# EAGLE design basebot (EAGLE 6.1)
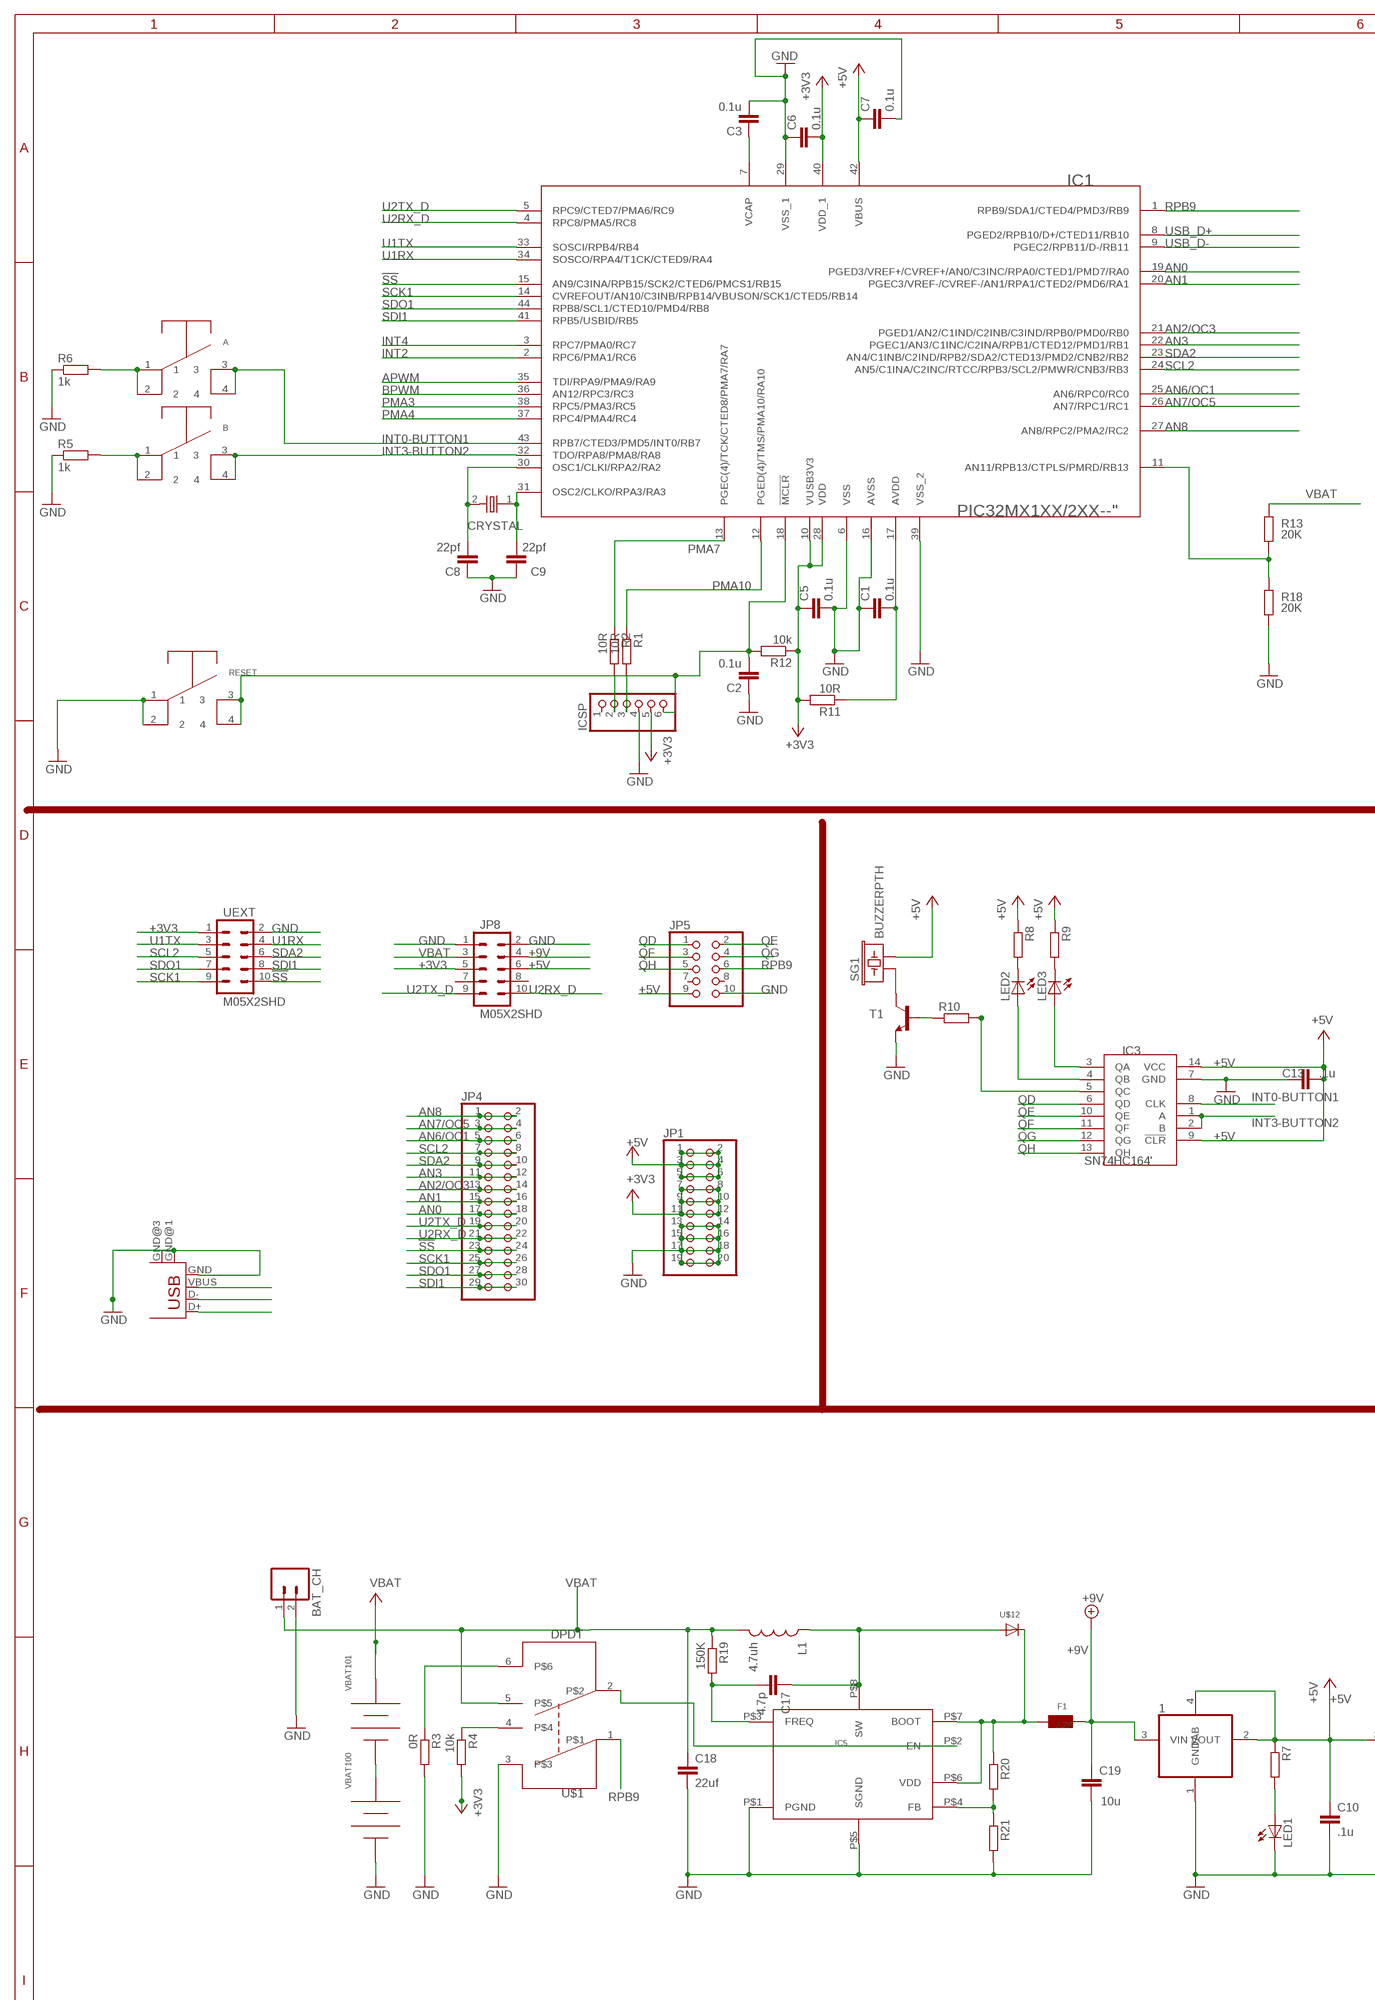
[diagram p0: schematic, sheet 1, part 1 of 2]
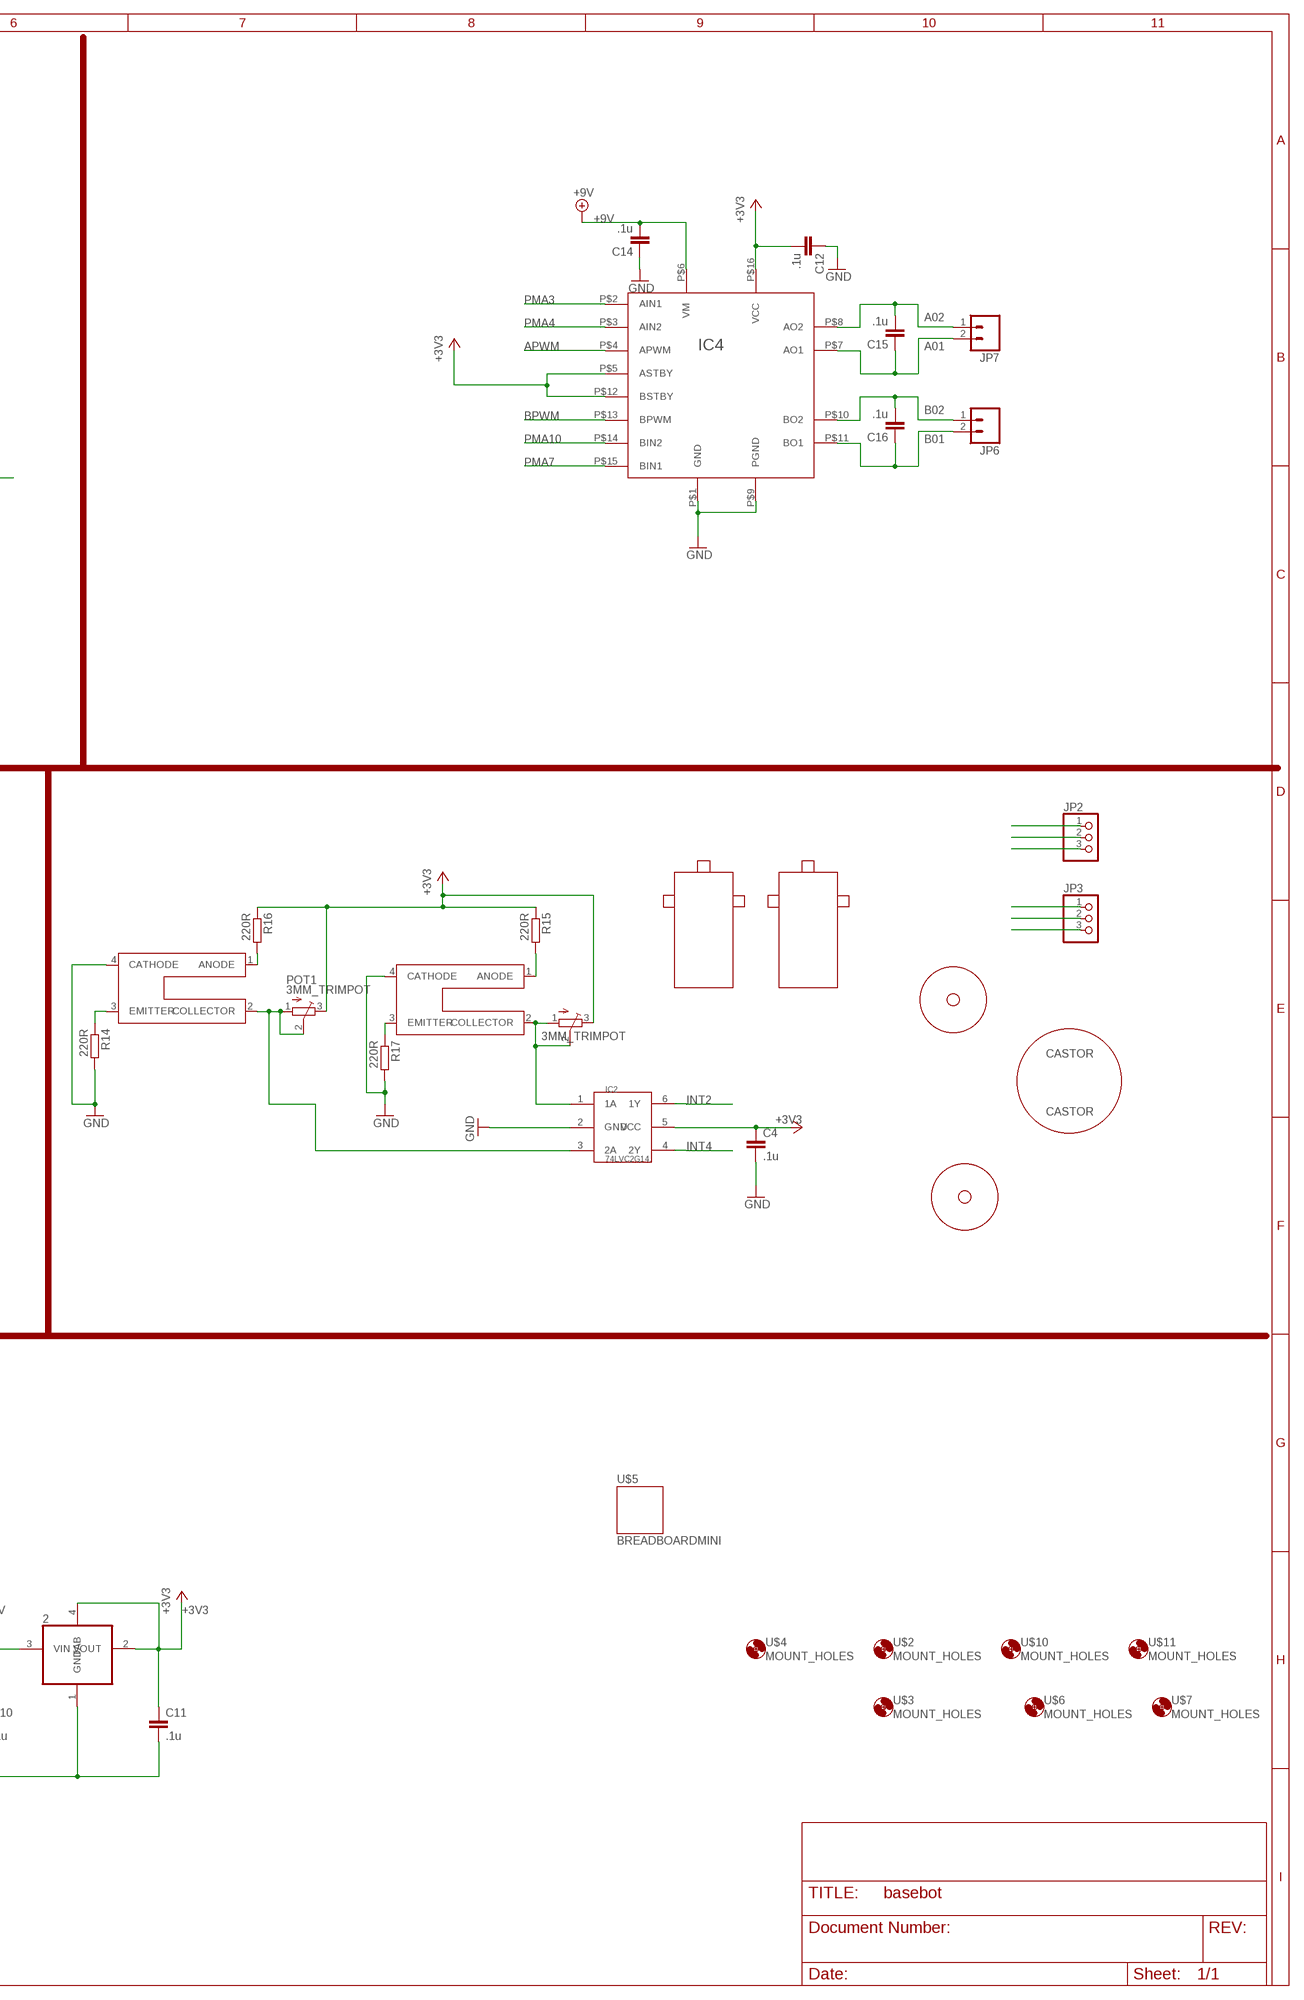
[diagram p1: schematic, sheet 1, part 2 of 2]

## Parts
1  REG1117  [SOT223]
2  REG1117  [SOT223]
A  SWITCH_MOMENTARY  [SWITCH_SMD]
B  SWITCH_MOMENTARY  [SWITCH_SMD]
BAT_CH  M02-JST-2-PTH-NO_SILK  [JST-2-PTH-NS]
C1  0.1u  C-EUC0805  [C0805]
C2  0.1u  C-EUC0805  [C0805]
C3  0.1u  C-EUC0805  [C0805]
C4  .1u  C-EUC0805  [C0805]
C5  0.1u  C-EUC0805  [C0805]
C6  0.1u  C-EUC0805  [C0805]
C7  0.1u  C-EUC0805  [C0805]
C8  22pf  C-EUC0805  [C0805]
C9  22pf  C-EUC0805  [C0805]
C10  .1u  C-EUC0805  [C0805]
C11  .1u  C-EUC0805  [C0805]
C12  .1u  C-EUC0805  [C0805]
C13  .1u  C-EUC0805  [C0805]
C14  .1u  C-EUC0805  [C0805]
C15  .1u  C-EUC0805  [C0805]
C16  .1u  C-EUC0805  [C0805]
C17  4.7p  C-EUC0805  [C0805]
C18  22uf  C-EUC0805  [C0805]
C19  10u  C-EUC0805  [C0805]
CASTOR  CASTOR  [CASTOR-16.66MM]
CRYSTAL  CRYSTAL2PIN  [CRYSTAL-2PIN]
F1  1.2A  PPTC  [PPTC1812]
IC1  PIC32MX1XX/2XX--"  [44TQFP]
IC2  74LVC2G14.  [6TSOP]
IC3  SN74HC164'  [SOIC-14]
IC4  TB6552FN  [16PIN_SSOP]
IC5  LM2623  [MSOP-8L-EDP]
ICSP  PINHD-1X6  [1X06]
JP1  PINHD-2X10  [2X10]
JP2  PINHD-1X3  [1X03]
JP3  PINHD-1X3  [1X03]
JP4  PINHD-2X15  [2X15]
JP5  PINHD-2X5  [2X05]
JP6  M02-JST-2-PTH-NO_SILK  [JST-2-PTH-NS]
JP7  M02-JST-2-PTH-NO_SILK  [JST-2-PTH-NS]
JP8  M05X2SHD  [2X5-SHROUDED]
L1  4.7uh  INDUCTORNPI75  [NPI75C]
LED1  LEDCHIP-LED0805  [CHIP-LED0805]
LED2  LEDCHIP-LED0805  [CHIP-LED0805]
LED3  LEDCHIP-LED0805  [CHIP-LED0805]
LEFT1  DUAL_SHAFT_PLASTIC_GEAR_MOTOR_ST1_LEFT  [DUAL_SHAFT_PLASTIC_GEAR_MOTOR_ST1_LEFT]
POT  3MM_TRIMPOT  [3MM_TRIMPOT]
POT1  3MM_TRIMPOT  [3MM_TRIMPOT]
R1  10R  R-EU_R0805  [R0805]
R2  10R  R-EU_R0805  [R0805]
R3  0R  R-EU_R0805  [R0805]
R4  10k  R-EU_R0805  [R0805]
R5  1k  R-EU_R0805  [R0805]
R6  1k  R-EU_R0805  [R0805]
R7  R-EU_R0805  [R0805]
R8  R-EU_R0805  [R0805]
R9  R-EU_R0805  [R0805]
R10  R-EU_R0805  [R0805]
R11  10R  R-EU_R0805  [R0805]
R12  10k  R-EU_R0805  [R0805]
R13  20K  R-EU_R0805  [R0805]
R14  220R  R-EU_R0805  [R0805]
R15  220R  R-EU_R0805  [R0805]
R16  220R  R-EU_R0805  [R0805]
R17  220R  R-EU_R0805  [R0805]
R18  20K  R-EU_R0805  [R0805]
R19  150K  R-EU_R0805  [R0805]
R20  R-EU_R0805  [R0805]
R21  R-EU_R0805  [R0805]
RESET  SWITCH_MOMENTARY  [SWITCH_SMD]
RIGHT1  DUAL_SHAFT_PLASTIC_GEAR_MOTOR_ST1_RIGHT  [DUAL_SHAFT_PLASTIC_GEAR_MOTOR_ST1_RIGHT]
SG1  BUZZERPTH  [BUZZER-12MM]
T1  MMBT2222ALT1-NPN-SOT23-BEC  [SOT23-BEC]
U$1  DPDT  [DPDT]
U$2  MOUNT_HOLES  [HOLES-1.6MM]
U$3  MOUNT_HOLES  [HOLES-1.6MM]
U$4  MOUNT_HOLES  [HOLES-1.6MM]
U$5  BREADBOARDMINI  [BREADBOARD-MINI]
U$6  MOUNT_HOLES  [HOLES-1.6MM]
U$7  MOUNT_HOLES  [HOLES-1.6MM]
U$8  GP1S092HCPIF  [GP1S092HCPIF]
U$9  GP1S092HCPIF  [GP1S092HCPIF]
U$10  MOUNT_HOLES  [HOLES-1.6MM]
U$11  MOUNT_HOLES  [HOLES-1.6MM]
U$12  DIODESMA  [SMADIODE]
UEXT  M05X2SHD  [2X5-SHROUDED]
USB1  USB-MB-S  [USB-MB-S]
VBAT100  BATTERY_HOLDERAA  [AA_BATTERY_HOLDER]
VBAT101  BATTERY_HOLDERAA  [AA_BATTERY_HOLDER]
WHEEL1  69X8MM-WHEEL  [69X8MM-WHEEL]
WHEEL2  69X8MM-WHEEL  [69X8MM-WHEEL]

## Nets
!SS: IC1.15(AN9/C3INA/RPB15/SCK2/CTED6/PMCS1/RB15) JP4.23 JP4.24 UEXT.10
+3V3: 2.2(VOUT) 2.4(TAB) C4.1 C5.1 C6.2 C11.1 C12.2 IC1.10(VUSB3V3) IC1.28(VDD) IC1.40(VDD_1) IC2.5(VCC) IC4.P$5(ASTBY) IC4.P$12(BSTBY) IC4.P$16(VCC) ICSP.5 JP1.7 JP1.8 JP1.9 JP1.10 JP1.11 JP1.12 JP8.5 POT1.3(E) POT.3(E) R4.2 R11.2 R12.1 R15.1 R16.1 UEXT.1
+5V: 1.2(VOUT) 1.4(TAB) 2.3(VIN) C7.1 C10.1 C13.1 IC1.42(VBUS) IC3.9(!CLR) IC3.14(VCC) JP1.1 JP1.2 JP1.3 JP1.4 JP1.5 JP1.6 JP2.2 JP3.2 JP5.9 JP8.6 R7.1 R8.1 R9.1 SG1.- USB1.VBUS
+9V: 1.3(VIN) C14.2 C19.2 F1.P$2 IC4.P$6(VM) JP8.4
A01: C15.1 IC4.P$7(AO1) JP7.2
A02: C15.2 IC4.P$8(AO2) JP7.1
AN0: IC1.19(PGED3/VREF+/CVREF+/AN0/C3INC/RPA0/CTED1/PMD7/RA0) JP4.17 JP4.18
AN1: IC1.20(PGEC3/VREF-/CVREF-/AN1/RPA1/CTED2/PMD6/RA1) JP4.15 JP4.16
AN2/OC3: IC1.21(PGED1/AN2/C1IND/C2INB/C3IND/RPB0/PMD0/RB0) JP4.13 JP4.14
AN3: IC1.22(PGEC1/AN3/C1INC/C2INA/RPB1/CTED12/PMD1/RB1) JP4.11 JP4.12
AN6/OC1: IC1.25(AN6/RPC0/RC0) JP2.1 JP4.5 JP4.6
AN7/OC5: IC1.26(AN7/RPC1/RC1) JP3.1 JP4.3 JP4.4
AN8: IC1.27(AN8/RPC2/PMA2/RC2) JP4.1 JP4.2
APWM: IC1.35(TDI/RPA9/PMA9/RA9) IC4.P$4(APWM)
B01: C16.1 IC4.P$11(BO1) JP6.2
B02: C16.2 IC4.P$10(BO2) JP6.1
BPWM: IC1.36(AN12/RPC3/RC3) IC4.P$13(BPWM)
GND: 1.1(GND) 2.1(GND) BAT_CH.2 C1.1 C2.1 C3.2 C4.2 C5.2 C6.1 C7.2 C8.1 C9.1 C10.2 C11.2 C12.1 C13.2 C14.1 C18.2 C19.1 IC1.6(VSS) IC1.16(AVSS) IC1.29(VSS_1) IC1.39(VSS_2) IC2.2(GND) IC3.7(GND) IC4.P$1(GND) IC4.P$9(PGND) IC5.P$1(PGND) IC5.P$5(SGND) ICSP.4 JP1.13 JP1.14 JP1.15 JP1.16 JP1.17 JP1.18 JP1.19 JP1.20 JP2.3 JP3.3 JP5.10 JP8.1 JP8.2 LED1.C R3.2 R5.1 R6.1 R14.2 R17.2 R18.2 R21.2 RESET.1 RESET.2 T1.E U$1.3 U$8.4(CATHODE) U$9.4(CATHODE) UEXT.2 USB1.GND USB1.GND@1(GND) USB1.GND@3(GND) VBAT100.-
INT0-BUTTON1: A.3 A.4 IC1.43(RPB7/CTED3/PMD5/INT0/RB7) IC3.8(CLK)
INT2: IC1.2(RPC6/PMA1/RC6) IC2.6(1Y)
INT3-BUTTON2: B.3 B.4 IC1.32(TDO/RPA8/PMA8/RA8) IC3.1(A) IC3.2(B)
INT4: IC1.3(RPC7/PMA0/RC7) IC2.4(2Y)
MCLR: C2.2 IC1.18(!MCLR) ICSP.6 R12.2 RESET.3 RESET.4
N$1: IC1.11(AN11/RPB13/CTPLS/PMRD/RB13) R13.2 R18.1
N$3: C3.1 IC1.7(VCAP)
N$5: C17.2 IC5.P$3(FREQ) R19.2
N$6: LED1.A R7.2
N$7: IC3.3(QA) LED3.A
N$8: IC3.4(QB) LED2.A
N$14: IC3.5(QC) R10.2
N$15: LED3.C R9.2
N$16: LED2.C R8.2
N$17: R10.1 T1.B
N$18: ICSP.3 R1.2
N$19: ICSP.2 R2.2
N$20: VBAT100.+ VBAT101.-
N$22: A.1 A.2 R6.2
N$23: B.1 B.2 R5.2
N$24: R4.1 U$1.4
N$25: R3.1 U$1.6
N$26: SG1.+ T1.C
N$27: C17.1 IC5.P$8(SW) L1.1 U$12.A
N$28: IC5.P$2(EN) U$1.2
N$29: IC5.P$4(FB) R20.2 R21.1
N$30: F1.P$1 IC5.P$6(VDD) IC5.P$7(BOOT) R20.1 U$12.C
N$36: R16.2 U$9.1(ANODE)
N$37: R15.2 U$8.1(ANODE)
N$38: R14.1 U$9.3(EMITTER)
N$39: C8.2 CRYSTAL.2 IC1.30(OSC1/CLKI/RPA2/RA2)
N$40: R17.1 U$8.3(EMITTER)
N$41: C9.2 CRYSTAL.1 IC1.31(OSC2/CLKO/RPA3/RA3)
N$42: IC2.3(2A) POT1.1(A) POT1.2(S) U$9.2(COLLECTOR)
N$44: C1.2 IC1.17(AVDD) R11.1
N$45: IC2.1(1A) POT.1(A) POT.2(S) U$8.2(COLLECTOR)
PMA3: IC1.38(RPC5/PMA3/RC5) IC4.P$2(AIN1)
PMA4: IC1.37(RPC4/PMA4/RC4) IC4.P$3(AIN2)
PMA7: IC1.13(PGEC(4)/TCK/CTED8/PMA7/RA7) IC4.P$15(BIN1) R2.1
PMA10: IC1.12(PGED(4)/TMS/PMA10/RA10) IC4.P$14(BIN2) R1.1
QD: IC3.6(QD) JP5.1
QE: IC3.10(QE) JP5.2
QF: IC3.11(QF) JP5.3
QG: IC3.12(QG) JP5.4
QH: IC3.13(QH) JP5.5
RPB9: IC1.1(RPB9/SDA1/CTED4/PMD3/RB9) JP5.6 U$1.1
SCK1: IC1.14(CVREFOUT/AN10/C3INB/RPB14/VBUSON/SCK1/CTED5/RB14) JP4.25 JP4.26 UEXT.9
SCL2: IC1.24(AN5/C1INA/C2INC/RTCC/RPB3/SCL2/PMWR/CNB3/RB3) JP4.7 JP4.8 UEXT.5
SDA2: IC1.23(AN4/C1INB/C2IND/RPB2/SDA2/CTED13/PMD2/CNB2/RB2) JP4.9 JP4.10 UEXT.6
SDI1: IC1.41(RPB5/USBID/RB5) JP4.29 JP4.30 UEXT.8
SDO1: IC1.44(RPB8/SCL1/CTED10/PMD4/RB8) JP4.27 JP4.28 UEXT.7
U1RX: IC1.34(SOSCO/RPA4/T1CK/CTED9/RA4) UEXT.4
U1TX: IC1.33(SOSCI/RPB4/RB4) UEXT.3
U2RX_D: IC1.4(RPC8/PMA5/RC8) JP4.21 JP4.22 JP8.10
U2TX_D: IC1.5(RPC9/CTED7/PMA6/RC9) JP4.19 JP4.20 JP8.9
USB_D+: IC1.8(PGED2/RPB10/D+/CTED11/RB10) USB1.D+
USB_D-: IC1.9(PGEC2/RPB11/D-/RB11) USB1.D-
VBAT: BAT_CH.1 C18.1 JP8.3 L1.2 R13.1 R19.1 U$1.5 VBAT101.+
Unconnected: ICSP.1 JP5.7 JP5.8 JP8.7 JP8.8

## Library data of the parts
1 2 = BaseApp:REG1117: 800mA and 1A Low Dropout (LDO) Positive Regulator 1.8V, 2.5V, 2.85V, 3.3V, 5V, and Adj http://www.digikey.com/product-detail/en/LM1117MPX-3.3%2FNOPB/LM1117MPX-3.3CT-ND/1010516
A B RESET = BaseApp:SWITCH_MOMENTARY: Soft Switch http://www.digikey.com/product-detail/en/EVQ-Q2B03W/P12932SCT-ND/762922
BAT_CH JP6 JP7 = SparkFun:M02: Header 2
C1-C19 = rcl:C-EU: CAPACITOR, European symbol
CASTOR = BaseApp:CASTOR
CRYSTAL = BaseApp:CRYSTAL: CRYSTAL
F1 = BaseApp:PPTC: PPTC FUSE :- Ih-750ma; It-1.5A; Vmax-40V
IC1 = BaseApp:PIC32MX1XX/2XX--: PIC32MX250F128D-I/PT http://www.digikey.com/product-detail/en/PIC32MX250F128D-I%2FPT/PIC32MX250F128D-I%2FPT-ND/3046589
IC2 = BaseApp:74LVC2G14: 74LVC2G14 :-Dual inverting Schmitt trigger http://www.digikey.com/product-detail/en/74LVC2G14GW,125/568-4840-1-ND/2116536
IC3 = BaseApp:SN74HC164: http://www.digikey.com/product-detail/en/SN74HC164PWR/296-14020-1-ND/522545 http://www.digikey.com/product-detail/en/MC74HC164ADG/MC74HC164ADGOS-ND/1479883
IC4 = BaseApp:TB6552FN
IC5 = BaseApp:LM2623: LM2623 http://www.digikey.com/product-detail/en/LM2623MM%2FNOPB/LM2623MM%2FNOPBCT-ND/483063
ICSP = adafruit:PINHD-1X6: PIN HEADER
JP1 = pinhead:PINHD-2X10: PIN HEADER
JP2 JP3 = adafruit:PINHD-1X3: PIN HEADER
JP4 = pinhead:PINHD-2X15: PIN HEADER
JP5 = pinhead:PINHD-2X5: PIN HEADER
JP8 UEXT = SparkFun:M05X2: Header 5x2 Standard 10-pin dual row 0.1" header. Commonly used with AVR-ISP. Use with Spark Fun Electronics SKU: PRT-00778
L1 = SparkFun:INDUCTOR: Inductors
LED1-LED3 = adafruit:LED: LED
LEFT1 = BaseApp:DUAL_SHAFT_PLASTIC_GEAR_MOTOR_ST1_LEFT
POT POT1 = BaseApp:3MM_TRIMPOT
R1-R21 = rcl:R-EU_: RESISTOR, European symbol
RIGHT1 = BaseApp:DUAL_SHAFT_PLASTIC_GEAR_MOTOR_ST1_RIGHT
SG1 = SparkFun:BUZZER: Buzzer 12mm
T1 = transistor:*-NPN-: NPN Transistror BF959 corrected 2008.03.06
U$1 = BaseApp:DPDT: http://www.digikey.com/product-detail/en/JS202011SCQN/401-2002-1-ND/1640098
U$2-U$4 U$6 U$7 U$10 U$11 = BaseApp:MOUNT_HOLES
U$5 = SparkFun:BREADBOARD: Breadboard Mini Self Adhesive
U$8 U$9 = BaseApp:GP1S092HCPIF: GP1S092HCPIF :- SMT, Gap : 2mm, Slit : 0.3mm Phototransistor Output, Compact Transmissive Photointerrupter
U$12 = BaseApp:DIODE
USB1 = con-usb-2(1):USB: USB Connectors
VBAT100 VBAT101 = BaseApp:BATTERY_HOLDER: BU2032SM-HD-G
WHEEL1 WHEEL2 = BaseApp:69X8MM-WHEEL

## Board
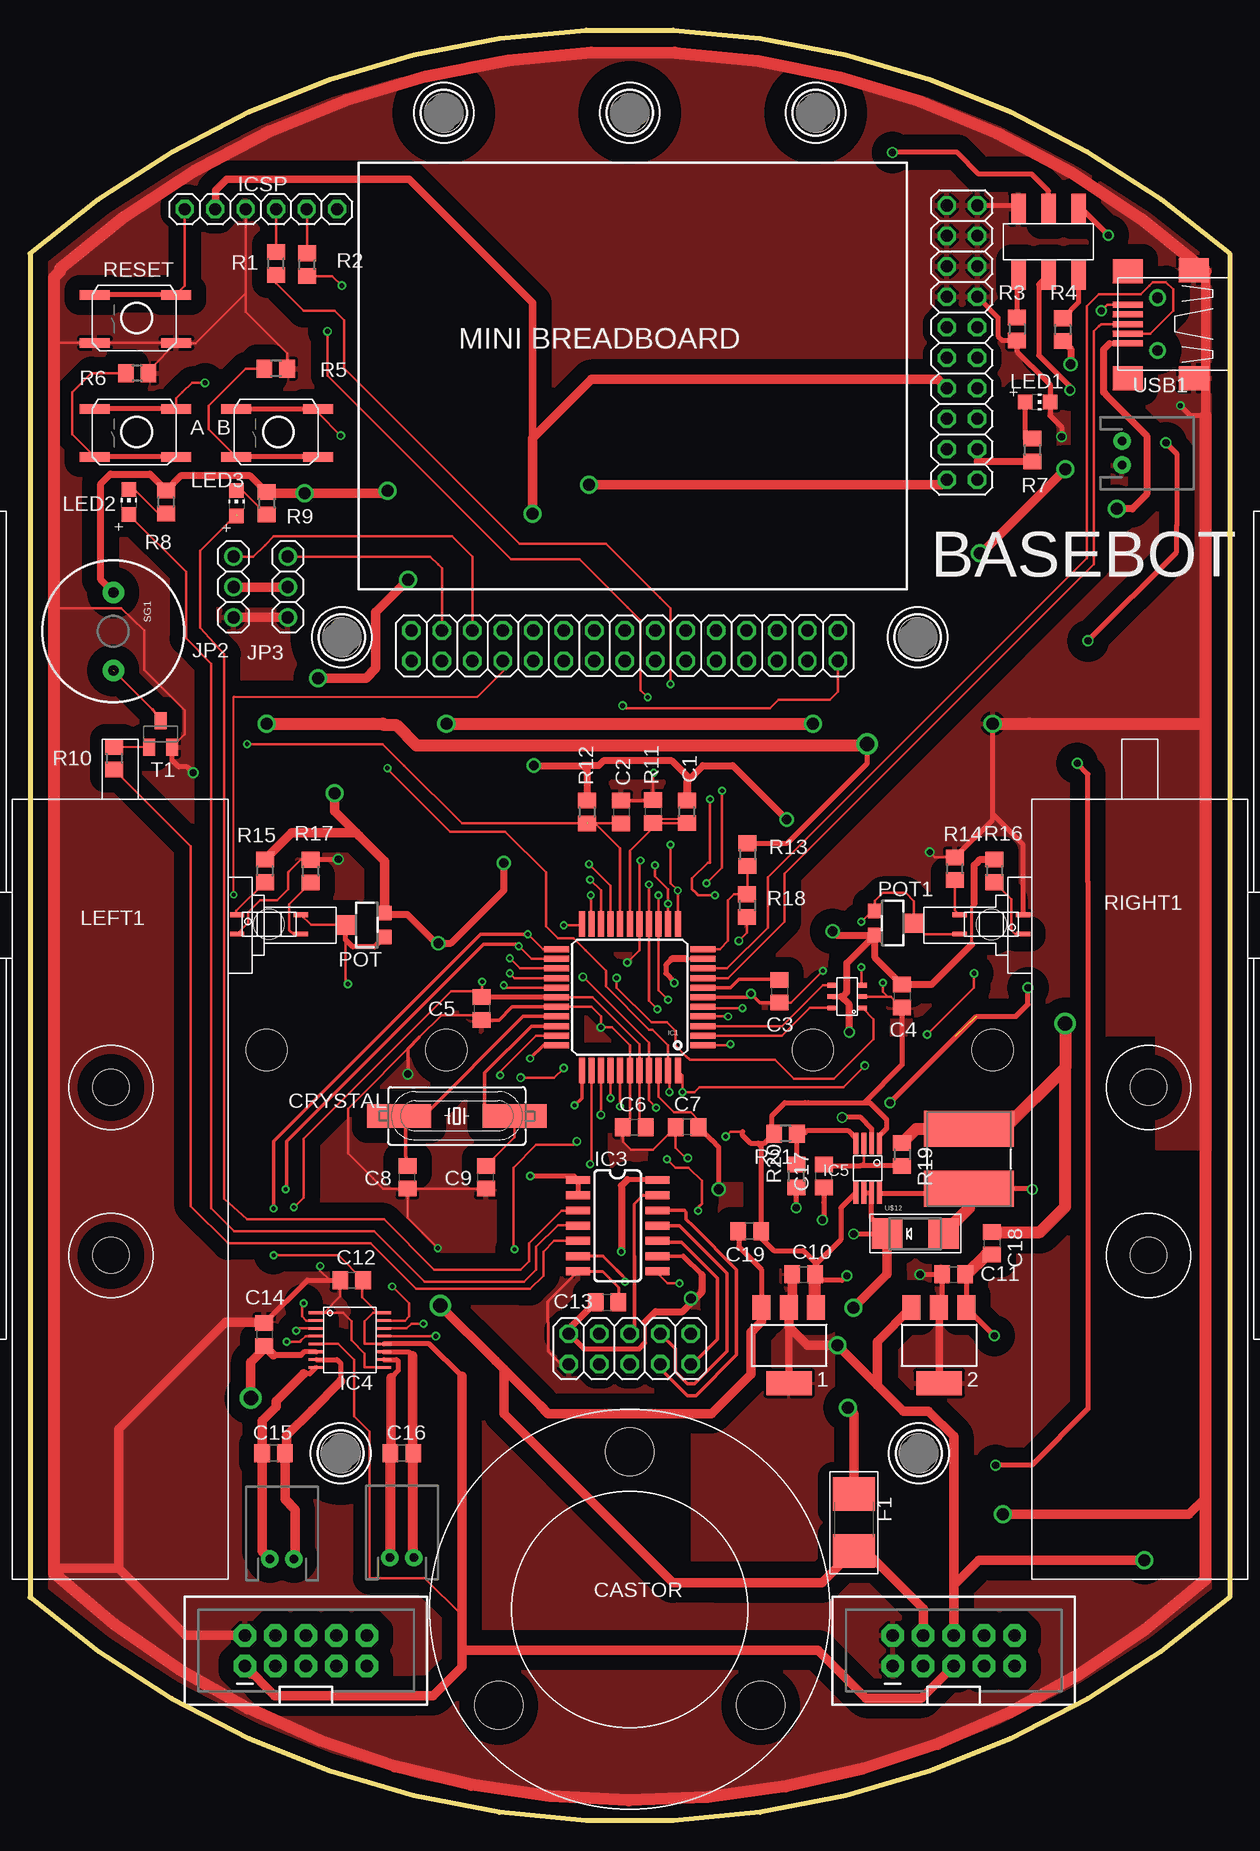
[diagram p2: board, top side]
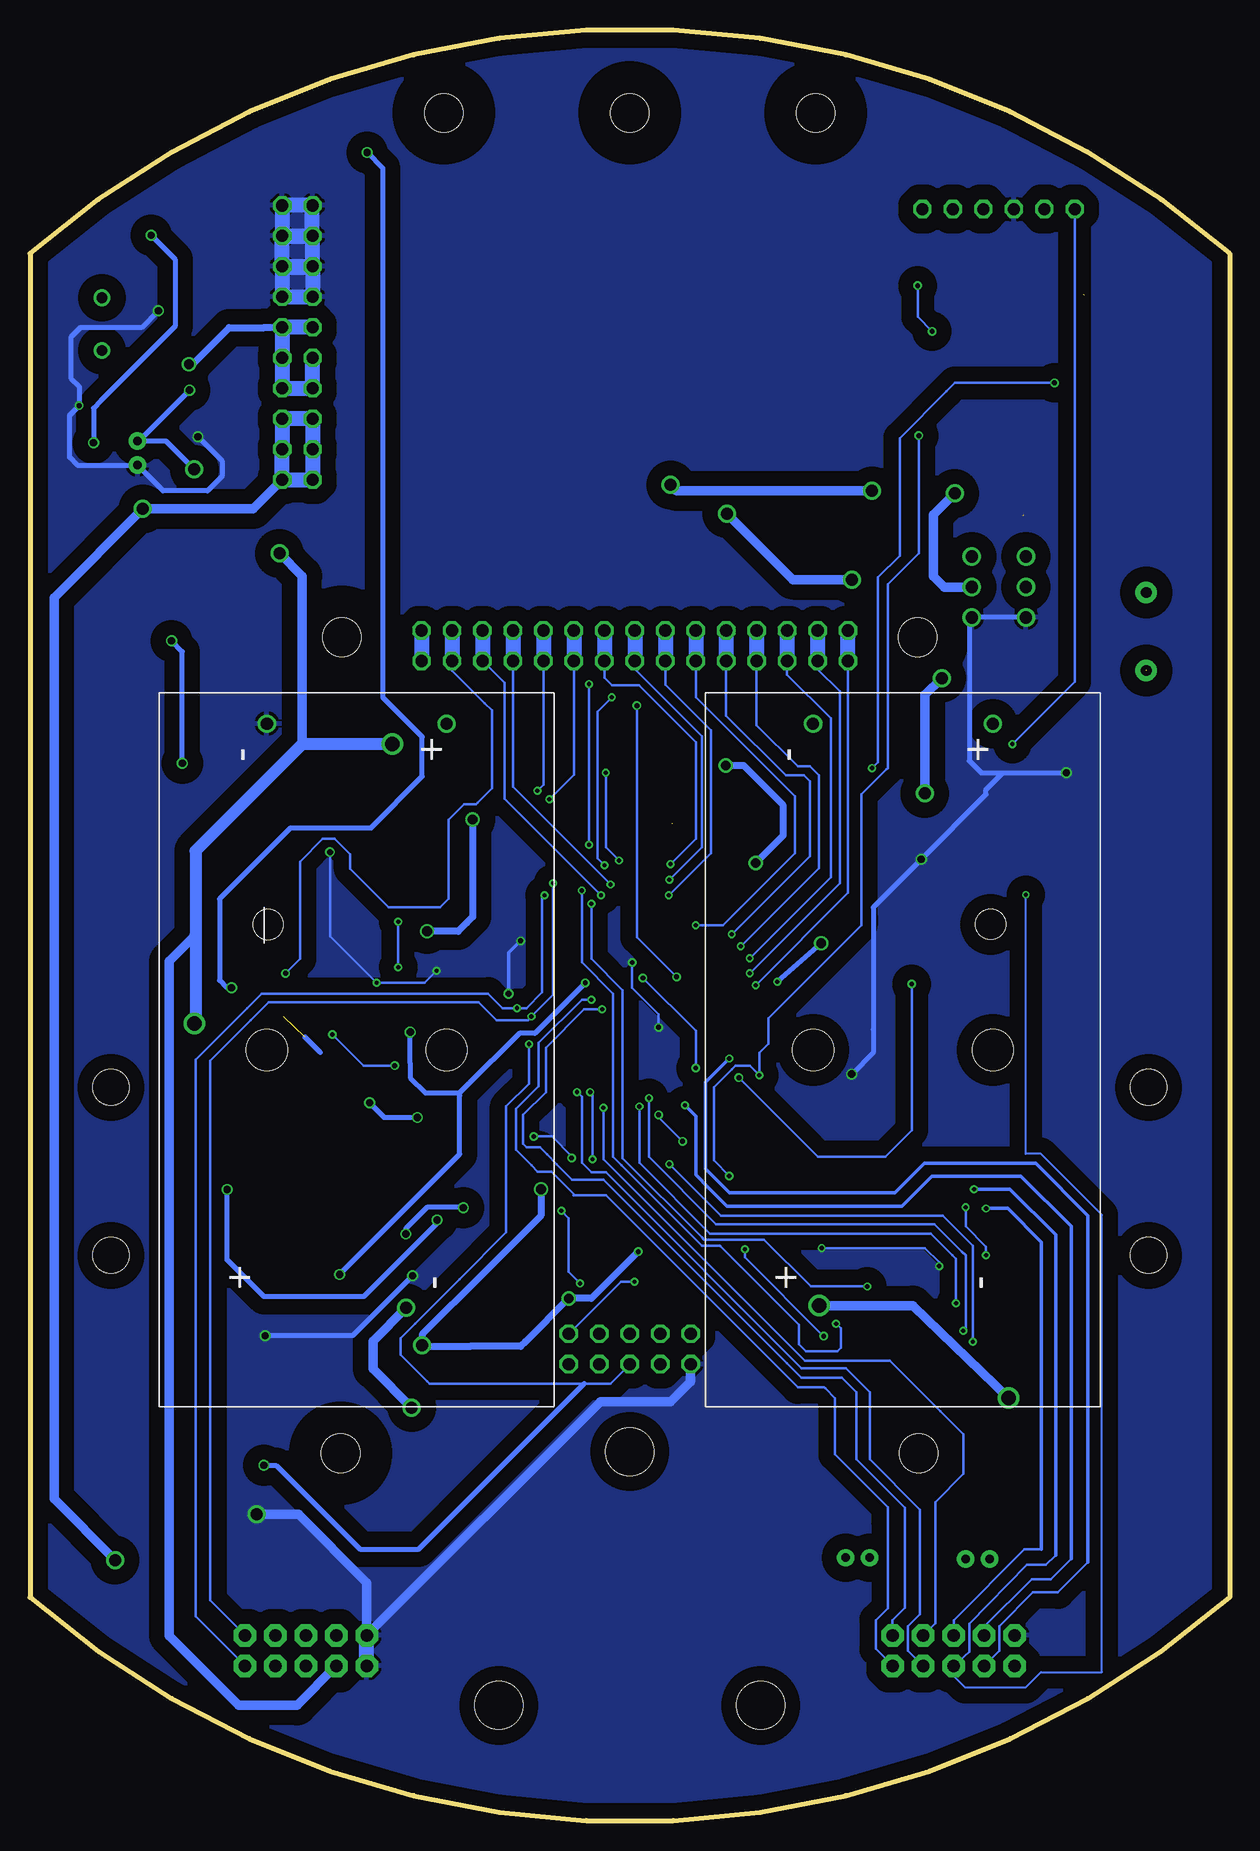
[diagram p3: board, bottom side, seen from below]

Size 100 x 149.22 mm. Coordinates in mm from the lower left corner, seen from the top.
Outline: 0,130.61 0,18.61 arc82 100,18.61 100,130.61 arc82 0,130.61
Copper layers (1*16): Top 0.035mm / dielectric 1.5mm / Bottom 0.035mm
Design rules: minimum track width 6mil, minimum drill 12mil, track to track 6mil, track to pad 6mil, pad to pad 6mil, via to via 6mil, smd to smd 0mil, copper to edge 10mil, drill to drill 10mil, minimum pad ring 10mil, minimum via ring 6mil, stop-mask expansion 2mil, vias tented up to drill 100mil, thermal gap 10mil

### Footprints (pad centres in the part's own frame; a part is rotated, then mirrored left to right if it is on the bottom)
SOT223 = smd 1.499 x 2.007: 1 -2.261,-3.15; 2 0.025,-3.15; 3 2.311,-3.15 | smd 3.81 x 2.007: 4 0,3.15
SWITCH_SMD = smd 2.5 x 0.762: 1 -2.54,2.73; 2 4.26,2.73; 3 -2.54,-1.27; 4 4.26,-1.27
JST-2-PTH-NS = drill 0.7 pad 1.448: 1 -1,0; 2 1,0
C0805 = smd 1.3 x 1.5: 1 -0.95,0; 2 0.95,0
CASTOR-16.66MM = hole 4: 0,13.13; 10.91,-8; -10.91,-8
CRYSTAL-2PIN = smd 5.334 x 1.93: 1 -4.826,0; 2 4.826,0
PPTC1812 = smd 2.78 x 3.5: P$1 -2.115,0; P$2 2.615,0
44TQFP = smd 2.1 x 0.5: 1 -6.1,4; 2 -6.1,3.2; 3 -6.1,2.4; 4 -6.1,1.6; 5 -6.1,0.8; 6 -6.1,0; 7 -6.1,-0.8; 8 -6.1,-1.6; 9 -6.1,-2.4; 10 -6.1,-3.2; 11 -6.1,-4; 23 6.1,-4; 24 6.1,-3.2; 25 6.1,-2.4; 26 6.1,-1.6; 27 6.1,-0.8; 28 6.1,0; 29 6.1,0.8; 30 6.1,1.6; 31 6.1,2.4; 32 6.1,3.2; 33 6.1,4 | smd 0.5 x 2.1: 12 -4,-6.1; 13 -3.2,-6.1; 14 -2.4,-6.1; 15 -1.6,-6.1; 16 -0.8,-6.1; 17 0,-6.1; 18 0.8,-6.1; 19 1.6,-6.1; 20 2.4,-6.1; 21 3.2,-6.1; 22 4,-6.1; 34 4,6.1; 35 3.2,6.1; 36 2.4,6.1; 37 1.6,6.1; 38 0.8,6.1; 39 0,6.1; 40 -0.8,6.1; 41 -1.6,6.1; 42 -2.4,6.1; 43 -3.2,6.1; 44 -4,6.1
6TSOP = smd 0.4 x 0.8: 1 0.6,-0.4; 2 1.55,-0.4; 3 2.5,-0.4; 4 2.5,2.1; 5 1.55,2.1; 6 0.6,2.1
SOIC-14 = smd 0.66 x 2.032: 1 -3.175,-3.315; 2 -1.905,-3.315; 3 -0.635,-3.315; 4 0.635,-3.315; 5 1.905,-3.315; 6 3.175,-3.315; 7 4.445,-3.315; 8 4.445,3.315; 9 3.175,3.315; 10 1.905,3.315; 11 0.635,3.315; 12 -0.635,3.315; 13 -1.905,3.315; 14 -3.175,3.315
16PIN_SSOP = smd 0.22 x 1.25: P$1 -2.2,-2.6; P$2 -1.55,-2.6; P$3 -0.9,-2.6; P$4 -0.25,-2.6; P$5 0.4,-2.6; P$6 1.05,-2.6; P$7 1.7,-2.6; P$8 2.35,-2.6; P$9 2.35,3.02; P$10 1.7,3.02; P$11 1.05,3.02; P$12 0.4,3.02; P$13 -0.25,3.02; P$14 -0.9,3.02; P$15 -1.55,3.02; P$16 -2.2,3.02
MSOP-8L-EDP = smd 0.4 x 1.8: P$1 -1,-1.9; P$2 -0.35,-1.9; P$3 0.3,-1.9; P$4 0.95,-1.9; P$5 0.95,2.2; P$6 0.3,2.2; P$7 -0.35,2.2; P$8 -1,2.2
1X06 = drill 1.016 octagon: 1 -6.35,0; 2 -3.81,0; 3 -1.27,0; 4 1.27,0; 5 3.81,0; 6 6.35,0
2X10 = drill 1.016 octagon: 1 -11.43,-1.27; 2 -11.43,1.27; 3 -8.89,-1.27; 4 -8.89,1.27; 5 -6.35,-1.27; 6 -6.35,1.27; 7 -3.81,-1.27; 8 -3.81,1.27; 9 -1.27,-1.27; 10 -1.27,1.27; 11 1.27,-1.27; 12 1.27,1.27; 13 3.81,-1.27; 14 3.81,1.27; 15 6.35,-1.27; 16 6.35,1.27; 17 8.89,-1.27; 18 8.89,1.27; 19 11.43,-1.27; 20 11.43,1.27
1X03 = drill 1.016: 1 -2.54,0; 2 0,0; 3 2.54,0
2X15 = drill 1.016 octagon: 1 -17.78,-1.27; 2 -17.78,1.27; 3 -15.24,-1.27; 4 -15.24,1.27; 5 -12.7,-1.27; 6 -12.7,1.27; 7 -10.16,-1.27; 8 -10.16,1.27; 9 -7.62,-1.27; 10 -7.62,1.27; 11 -5.08,-1.27; 12 -5.08,1.27; 13 -2.54,-1.27; 14 -2.54,1.27; 15 0,-1.27; 16 0,1.27; 17 2.54,-1.27; 18 2.54,1.27; 19 5.08,-1.27; 20 5.08,1.27; 21 7.62,-1.27; 22 7.62,1.27; 23 10.16,-1.27; 24 10.16,1.27; 25 12.7,-1.27; 26 12.7,1.27; 27 15.24,-1.27; 28 15.24,1.27; 29 17.78,-1.27; 30 17.78,1.27
2X05 = drill 1.016 octagon: 1 -5.08,-1.27; 2 -5.08,1.27; 3 -2.54,-1.27; 4 -2.54,1.27; 5 0,-1.27; 6 0,1.27; 7 2.54,-1.27; 8 2.54,1.27; 9 5.08,-1.27; 10 5.08,1.27
2X5-SHROUDED = drill 1.016 pad 1.88 octagon: 1 -1.27,5.08; 2 1.27,5.08; 3 -1.27,2.54; 4 1.27,2.54; 5 -1.27,0; 6 1.27,0; 7 -1.27,-2.54; 8 1.27,-2.54; 9 -1.27,-5.08; 10 1.27,-5.08
NPI75C = smd 3 x 7.5: 1 -2.5,0; 2 2.5,0
CHIP-LED0805 = smd 1.2 x 1.2: A 0,-1.05; C 0,1.05
DUAL_SHAFT_PLASTIC_GEAR_MOTOR_ST1_LEFT = hole 3: 12.75,-13.5; 12.75,-27.5
3MM_TRIMPOT = smd 1.2 x 1.2: 1 -1,-1.8; 3 1,-1.8 | smd 1.6 x 1.5: 2 0,1.45
R0805 = smd 1.3 x 1.5: 1 -0.95,0; 2 0.95,0
DUAL_SHAFT_PLASTIC_GEAR_MOTOR_ST1_RIGHT = hole 3: -12.75,-13.5; -12.75,-27.5
BUZZER-12MM = drill 0.9 pad 1.778: + 3.25,0; - -3.25,0
SOT23-BEC = smd 1 x 1.4: B -0.95,-1.1; C 0,1.1; E 0.95,-1.1
DPDT = smd 1.2 x 2.5: 1 0,1.25; 2 2.5,1.25; 3 5,1.25; 4 0,6.75; 5 2.5,6.75; 6 5,6.75
HOLES-1.6MM = hole 3.2: 0,0
GP1S092HCPIF = smd 1.2 x 0.4: 1 2.65,0.2; 2 -2.65,0.2; 3 -2.65,1.8; 4 2.65,1.8 | hole 2.5: 0,1
SMADIODE = smd 2.54 x 2.54: A 2.349,0; C -2.349,0
USB-MB-S = smd 2.5 x 0.5: D+ 2.5,0; D- 2.5,0.8; GND 2.5,-1.6; ID 2.5,-0.8; VBUS 2.5,1.6 | smd 2.5 x 2: GND@1 -3,4.5; GND@2 2.5,4.5; GND@3 -3,-4.5; GND@4 2.5,-4.4 | drill 0.9: P$5 0,2.2; P$6 0,-2.2
AA_BATTERY_HOLDER = drill 1.02: + 27.18,-7.5; - 27.18,7.49 | hole 3.43: 0,-7.5; 0,7.49

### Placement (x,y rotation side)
1  63.28,39.61 180 top
2  75.8,39.61 180 top
A  9.66,116.37 180 top
B  21.46,116.37 180 top
BAT_CH  91.04,113.96 270 top
C1  51.94,84.1 270 top
C2  49.29,84.05 270 top
C3  62.49,69.11 270 top
C4  72.7,68.71 270 top
C5  37.66,67.67 270 top
C6  50.38,57.8 0 top
C7  54.78,57.8 180 top
C8  31.46,53.61 90 top
C9  38,53.61 90 top
C10  64.5,45.51 0 top
C11  77,45.51 0 top
C12  26.82,45.05 0 top
C13  48.1,43.21 0 top
C14  19.54,40.51 270 top
C15  20.3,30.61 180 top
C16  31,30.61 180 top
C17  66.2,53.71 90 top
C18  80.2,48.11 270 top
C19  60,49.11 180 top
CASTOR  50,17.61 0 top
CRYSTAL  35.58,58.72 180 top
F1  68.67,25.09 270 top
IC1  50,68.61 180 top
IC2  68.98,67.12 90 top
IC3  49,50.21 270 top
IC4  26.47,40.12 270 top
IC5  69.81,54.52 180 top
ICSP  19.25,134.29 180 top
JP1  77.7,123.17 90 top
JP2  16.97,102.8 270 top
JP3  21.49,102.8 270 top
JP4  49.58,97.91 0 top
JP5  50,39.31 180 top
JP6  31,21.91 0 top
JP7  21,21.81 0 top
JP8  77,14.16 90 top
L1  78.29,55.14 90 top
LED1  84,118.21 270 top
LED2  8.24,109.88 0 top
LED3  17.22,109.78 0 top
LEFT1  -6,74.61 0 top
POT  27.76,74.64 90 top
POT1  72.24,74.79 270 top
R1  20.51,129.76 90 top
R2  23.11,129.66 90 top
R3  82.29,124.3 270 top
R4  86.09,124.25 270 top
R5  20.49,121 180 top
R6  8.94,120.62 180 top
R7  83.58,114.21 90 top
R8  11.34,109.88 270 top
R9  19.72,109.78 270 top
R10  7.02,88.53 270 top
R11  54.76,84.07 90 top
R12  46.44,84.05 270 top
R13  59.81,80.5 270 top
R14  77.11,79.32 90 top
R15  19.59,79.15 270 top
R16  80.39,79.15 270 top
R17  23.41,79.12 90 top
R18  59.79,76.25 270 top
R19  72.7,55.51 270 top
R20  63.9,53.71 90 top
R21  62.99,57.25 180 top
RESET  9.66,125.87 180 top
RIGHT1  106,74.61 0 top
SG1  6.95,99.1 270 top
T1  10.89,90.55 0 top
U$1  87.4,135.57 180 top
U$2  34.5,142.31 0 top
U$3  50,142.31 0 top
U$4  65.5,142.31 0 top
U$5  27.4,102.61 0 top
U$6  26,98.61 0 top
U$7  74,98.61 0 top
U$8  19.92,75.69 180 top
U$9  80.14,73.68 0 top
U$10  25.9,30.61 0 top
U$11  74.1,30.61 0 top
U$12  73.8,48.91 0 top
UEXT  23,14.16 90 top
USB1  94,124.71 180 top
VBAT100  72.77,64.23 90 bottom
VBAT101  27.23,64.23 90 bottom
WHEEL1  not placed on the board
WHEEL2  not placed on the board

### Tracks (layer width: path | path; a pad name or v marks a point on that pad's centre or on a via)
!SS  (via drill 0.35)
  Top 0.2: v51.6,78.01 IC1.15 51.6,68.31 v52.3,67.61
  Bottom 0.2: JP4.23 59.74,86.15 v51.6,78.01 | UEXT.10 28.1,15.45 28.1,16.71 27.08,17.73 27.08,25.69 27.08,26.09 31.1,30.11 31.1,35.71 32.3,36.91 35.7,36.91 36.9,38.11 52.2,53.41 54.6,53.41 54.8,53.41 56.1,54.71 56.9,55.51 57.5,56.11 58.6,56.11 58.9,56.41 58.9,58.31 58.9,58.81 57,60.71 57,64.41 53.8,67.61 v52.3,67.61
  Bottom 1.27: JP4.24 JP4.23
+3V3  (via drill 0.35, 0.4, 0.6, 0.8, 1)
  Top 0.2: C6.2 50.8,58.33 IC1.40 50.8,64.71 46.9,68.61 IC1.28 | IC4.P$12 27.9,39.72 27.9,41.61 28.61,42.32 IC4.P$16 28.99,42.32 27.7,43.61 27.7,44.98 C12.2 25.71,47.11 v20.3,47.11 | 27.45,82.06 27.2,82.31 | v37.7,69.91 37.7,69.11 | 37.7,69.11 37.7,68.61 C5.1 | 67.76,68.67 67.4,68.67 67.64,68.67 | IC1.10 54.7,71.81 | IC4.P$5 25.69,39.72 27,38.41 27,33.71 28.3,32.41 28.3,20.21 32.9,20.21 36,17.11 | 76.07,124.44 JP1.12 | 37.7,69.11 36.1,69.11 35.1,69.11 22.8,56.81 22.8,55.61 22.8,51.91 v22,51.11
  Top 0.25: 78.5,73.01 78.5,76.2 78.73,76.43
  Top 0.3: 54.8,85.06 R11.2
  Top 0.4: IC2.5 67.4,68.67 | 36,37.01 33.29,39.72 IC4.P$12 | 53.5,71.81 53,71.31 53,70.61 53.7,69.91 v53.7,69.81 | v74.2,45.51 C11.1
  Top 0.406: IC1.28 C5.1 | 2.2 76.05,43.03 C11.1
  Top 0.6: 54.8,85.06 54.8,87.01 53.5,88.31 47.8,88.31 47.4,87.91 46.1,87.91 | 78.5,73.01 75.15,69.66 C4.1 70.44,71.92 POT1.3 | 67.76,68.67 68.1,69.01 68.1,71.45 POT1.3 | 54.7,71.81 53.5,71.81 | v68.3,65.71 68.3,68.01 67.64,68.67 | v39.5,79.81 39.5,77.51 35.1,73.11 v34.04,73.11 33.86,73.11 31.46,75.52 29.68,75.52 POT.3 | v42,87.91 46.1,87.91 | R11.2 54.76,86.57 56.1,87.91 58.6,87.91 v63.1,83.41 | v66.9,74.11 67.22,73.79 POT1.3 | 46.1,87.91 46.44,87.57 R12.1 | R4.2 86.75,122.64 v86.75,121.36 | 78.73,76.43 78.73,79.62 78.88,79.78 79.2,80.1 R16.1
  Top 0.61: ICSP.5 15.5,134.34 15.5,135.86 16.41,136.78 31.61,136.78 41.9,126.48 41.9,114.89 | 2.2 75.8,42.76 2.4
  Top 0.8: POT.3 29.56,79.95 27.45,82.06 25.4,84.11 v25.4,85.61 | 27.2,82.31 21.8,82.31 R15.1 | JP8.5 74.32,10.21 69.7,10.21 65.7,14.21 36,14.21 | 18.6,12.21 arc-90 UEXT.1 20.4,10.41 32.1,10.41 33.6,10.41 36,12.81 36,14.21 | 36,14.21 36,17.11 36,37.01 | v41.9,108.91 41.9,114.89 41.9,115.21 46.8,120.11 74.65,120.11 75.68,120.11 JP1.8 | v31.5,103.41 28.8,100.71 28.8,96.01 28,95.21 v24,95.21
  Bottom 0.2: v20.3,47.11 20.3,47.81 22,49.51 v22,51.11
  Bottom 0.3: 80.5,124.41 80.47,124.44
  Bottom 0.4: v34.04,73.11 v37.7,69.91 | v53.7,69.81 57.9,65.61 59.2,65.61 59.6,65.21 63.34,61.47 64.17,60.64 | v68.3,65.71 68.3,63.11 68.3,62.61 68.3,61.91 67.03,60.64 64.17,60.64 | v74.2,45.51 64.17,55.54 64.17,60.44 64.17,60.64
  Bottom 0.6: 80.5,124.41 83.4,124.41 86.45,121.36 v86.75,121.36 | 80.47,124.44 JP1.11 | v39.5,79.81 37.2,82.11 37.2,84.61 40.5,87.91 v42,87.91 | v63.1,83.41 63.1,75.31 63.6,74.81 64.3,74.11 v66.9,74.11
  Bottom 0.8: v41.9,108.91 36.4,103.41 v31.5,103.41 | v24,95.21 25.4,93.81 v25.4,85.61
  Bottom 1.27: JP1.12 JP1.11 JP1.9 JP1.7 JP1.8 76.4,119.36 76.43,119.39 JP1.10
  pour Top (isolate 1.27): 82,60.61 72,60.61 72,26.61 90,26.61 90,60.61
+5V  (via drill 0.4, 0.8, 1)
  Top 0.2: IC1.42 52.4,60.31 53.7,59.01 55.1,59.01 55.73,58.38 C7.1 | 19.68,110.73 R9.1 19.84,110.61 | IC3.14 52.29,53.41
  Top 0.3: JP5.9 44.97,40.58 45,40.61 | IC3.9 53.98,47.03 54.48,47.03 | 51.26,39.81 51.26,41.51
  Top 0.4: JP5.9 46.19,39.31 50.8,39.31 51.26,39.81 | 11.34,110.87 R8.1 | 90,123.11 USB1.VBUS | C7.1 56.8,56.73 57.4,56.13 v57.4,52.61 | 54.48,47.03 56,45.51 | 52.29,53.41 49.8,53.41
  Top 0.6: 45,40.61 45,41.06 C13.1 | R8.1 12.62,112.11 14.6,112.11 18.3,112.11 19.68,110.73 | JP1.3 78.97,113.26 R7.1 | v90.6,109.31 91.9,109.31 93.1,110.51 93.1,115.41 89.8,118.71 89.5,119.01 89.5,121.31 89.5,122.61 90,123.11 | SG1.- 5.9,103.4 5.9,111.41 6.7,112.21 10,112.21 11.34,110.87 | 56,45.51 56,44.01 55.5,43.51 v55.1,43.51 55.1,43.11 54.4,42.41 52.16,42.41 51.26,41.51 | 49.8,53.41 49.3,52.91 v49.3,47.41
  Top 0.61: 1.4 63.26,36.46 1.2
  Top 0.8: C10.1 63.55,43.05 1.2 63.26,41.15 64.8,39.61 v67.3,39.61 70.64,36.27 | 77,19.61 77,32.01 74.9,34.11 72.8,34.11 70.64,36.27 | 77,19.61 JP8.6 77,19.61 | JP2.2 JP3.2 | 19.84,110.61 v22.9,110.61 29.6,110.61 v29.8,110.81 | v46.6,111.31 73.97,111.31 76,111.31 JP1.2 | 77,19.61 79.1,21.71 v92.9,21.71 | 2.3 70.64,39.91 70.64,36.27
  Bottom 0.4: v67.3,39.61 67.2,39.51
  Bottom 0.6: 58.7,39.91 v55.1,43.51 53.2,43.51 v49.3,47.41 | 58.7,39.91 59.1,39.51 63.3,39.51 67.2,39.51 | 57.5,41.11 58.7,39.91 | v57.4,52.61 57.4,50.41 62.2,45.61 67.3,40.51 v67.3,39.61
  Bottom 0.8: JP1.1 81.4,109.31 v90.6,109.31 98,101.91 98,68.51 98,26.81 v92.9,21.71 | JP3.2 23.79,102.8 24.7,103.71 24.7,108.81 v22.9,110.61 | v46.6,111.31 46.1,110.81 v29.8,110.81
  Bottom 1.27: JP1.1 JP1.2 | JP1.4 JP1.6 JP1.5 JP1.3 JP1.1 | JP1.1 76.4,111.74 76.4,114.21
  pour Top (isolate 1.27): 57.9,53.11 67,53.11 67,21.71 55.2,21.71 55.2,53.01 57.9,53.01
+9V  (via drill 1.2)
  Top 0.4: IC4.P$6 22.84,39.07 22.57,38.79 | C19.2 59.1,49.06 59.1,47.81 60.97,45.94 1.3
  Top 0.406: C14.2 19.4,39.56 19.4,39.21
  Top 0.508: 22.57,38.79 20.3,38.79
  Top 0.762: 20.3,38.79 C14.2
  Top 0.8: JP8.4 74.46,16.01 74.46,17.65 69.64,22.47 F1.P$2 66,19.81 59.1,19.81 57.3,19.81 53.6,19.81 39.5,33.91 39.5,37.61 38.8,38.31 | v18.4,35.21 18.4,38.21 19.4,39.21 19.7,39.51 | 1.3 60.97,41.58 60.3,40.91 60.1,40.71 60.1,37.21 56.8,33.91 46.8,33.91 43.2,33.91 42.5,34.61 38.8,38.31 | v34.2,42.91 38.8,38.31
  Bottom 0.8: v34.2,42.91 26.4,42.91 v18.4,35.21
A01
  Top 0.2: 21.4,32.11 21.4,31.91 | 21.4,30.76 C15.1
  Top 0.4: IC4.P$7 25.59,38.42 25.9,38.11 25.9,36.61
  Top 0.8: 25.9,36.61 23.5,34.21 21.4,32.11 | 21.4,31.91 21.4,30.76 | JP7.2 22.1,21.91 22.1,25.91 21.25,26.76 C15.1
A02
  Top 0.4: IC4.P$8 23.32,37.22 22.79,37.22
  Top 0.8: JP7.1 19.35,22.46 C15.2 19.35,33.25 19.35,33.32 20.51,34.48 20.51,34.94 22.79,37.22
AN0  (via drill 0.35)
  Top 0.2: IC1.19 48.4,77.91 v46.6,79.71
  Bottom 0.2: JP4.17 52.12,95.23 51.5,94.61 49.25,94.61 44.5,89.86 44.5,81.81 v46.6,79.71
  Bottom 1.27: JP4.18 JP4.17
AN1  (via drill 0.35)
  Top 0.2: IC1.20 47.6,77.51 v46.7,78.41
  Bottom 0.2: JP4.15 49.58,95.94 44,90.36 44,81.41 44,81.21 44,81.11 v46.7,78.41
  Bottom 1.27: JP4.16 JP4.15
AN2/OC3  (via drill 0.35)
  Top 0.2: IC1.21 46.75,74.76 v46.75,77.11
  Bottom 0.2: v46.75,77.11 43.25,80.61 43.25,90.86 47.04,94.65 JP4.13
  Bottom 1.27: JP4.14 JP4.13
AN3  (via drill 0.35)
  Top 0.2: IC1.22 45.9,74.61 v44.5,74.61
  Bottom 0.2: v44.5,74.61 42.25,74.61 36.25,80.61 36.25,85.36 44.5,93.61 JP4.11
  Bottom 1.27: JP4.12 JP4.11
AN6/OC1  (via drill 0.35)
  Top 0.2: IC1.25 40.85,71.01 v40,71.86 | JP2.1 17,105.31 18.6,105.31 19.59,106.29 20.3,107.01 29.05,107.01 35.2,107.01 36.88,105.33 JP4.6
  Bottom 0.2: v40,71.86 33.25,78.61 33.25,91.86 36.88,95.49 JP4.5
  Bottom 1.27: JP4.6 JP4.5
AN7/OC5  (via drill 0.35)
  Top 0.2: IC1.26 40.4,70.21 v40,70.61 | JP3.1 28.18,105.34 33.37,105.34 34,104.71 34.34,104.37 JP4.4
  Bottom 0.2: v40,70.61 32.5,78.11 32.5,94.11 34.34,95.95 JP4.3
  Bottom 1.27: JP4.4 JP4.3
AN8  (via drill 0.35)
  Top 0.2: IC1.27 39.7,69.41 v39.5,69.61
  Bottom 0.152: JP4.2 32.22,98.74 31.8,98.74
  Bottom 0.2: v39.5,69.61 31.8,77.31 JP4.1
  Bottom 1.27: JP4.1 31.8,98.74 JP4.2 31.8,99.31
APWM  (via drill 0.35)
  Top 0.2: v46.7,54.71 46.8,54.81 IC1.35 | IC4.P$4 22.96,40.37 22.6,40.01 22.5,39.91 v21.4,39.91
  Bottom 0.2: v21.4,39.91 21.4,47.91 23.9,50.41 42.4,50.41 v46.7,54.71
B01
  Top 0.4: IC4.P$11 31.58,39.07 31.91,38.74
  Top 0.8: 31.91,38.74 31.91,30.65 C16.1
  Top 0.813: JP6.2 31.95,21.96 C16.1
B02
  Top 0.254: 30.05,31.66 30.05,31.14 C16.2
  Top 0.4: IC4.P$10 30.56,38.42 30.7,38.28 30.7,37.52 30.09,36.91
  Top 0.8: 30.09,36.91 30.09,31.17 30.05,31.14
  Top 0.813: C16.2 30,30.56 JP6.1
BPWM  (via drill 0.35, 0.4)
  Top 0.2: IC4.P$13 v33.84,40.37 | v40.4,47.61 40.3,47.71 40.3,54.41 42.2,56.31 43.7,56.31 45.3,56.31 v45.6,56.61 | v47.6,58.81 IC1.36
  Bottom 0.2: v40.4,47.61 40.4,46.93 v33.84,40.37 | v45.6,56.61 47.6,58.61 v47.6,58.81
GND  (via drill 0.35, 0.4, 0.5, 0.6, 1)
  Top 0.2: 24.5,42.31 25.87,43.68 C12.1 25.83,45.01 25,45.01 24.2,45.81 v24.2,46.21 | 24.5,42.31 23.7,42.31 23.71,42.32 IC4.P$1 | v50.9,80.01 50.8,79.91 IC1.16 50.8,72.71 50.8,72.51 v49.8,71.51 | v52,87.31 51.94,87.25 C1.1 | U$8.4 18.2,74.82 18.2,75.71 19.2,76.71 20.6,76.71 21.5,77.61 21.5,78.21 21.5,79.01 21.6,79.11 22.56,80.07 R17.2 | U$9.4 82.7,75.57 | IC2.2 71.5,68.67 | 71.5,68.67 71.79,68.67 C4.2 | C4.2 72.74,67.72 | C3.2 63.45,68.16 v66.1,70.81 | v71.1,69.81 71.1,69.07 71.5,68.67 | 81.8,91.41 83.3,91.41 | IC1.29 46.8,67.81 47.6,67.01 v47.6,66.11 48.5,66.11 50,64.61 IC1.39 50,58.37 C6.1 49.43,56.58 50.1,55.91 51.94,55.91 C7.2 53.83,56.08 54.7,55.21 v54.85,55.21 | IC4.P$9 27.9,37.77 27.9,38.91 26.8,40.01 26.8,41.61 26.1,42.31 24.5,42.31 | C8.1 31.46,50.25 v34,47.71 | 2,123.31 2.17,123.14 RESET.2 RESET.1 | RESET.1 12.23,123.11 13.8,123.11 17.98,127.29 | 17.98,127.29 ICSP.4 | R6.1 9.99,120.62 10,120.61 10,120.94 RESET.1 | 17.98,127.29 17.98,125.73 21.44,122.27 R5.1 | T1.E 12.9,90.51 12.9,92.51 9.5,95.91 9.5,99.21 7.6,101.01 1.8,101.01 | C5.2 37.27,67.11 34.3,67.11 32.45,65.26 26.5,59.31 26.5,58.61 26.5,55.61 28.6,53.51 29.45,52.66 C8.1 | v58,57.01 58.4,57.41 59.4,57.41 | R18.2 59.79,74 v59.1,73.31 | v89.3,125.81 89.7,126.21 89.8,126.31 USB1.GND | v75,80.71 75.44,80.27 R14.2 | C9.1 C8.1 | 69.56,59.82 70.02,59.82 | 72.7,67.64 C4.2
  Top 0.254: JP5.10 44.27,38.04 43.2,39.11 43.2,41.5 43.2,43.28 IC3.7 47.74,45.76 48.4,45.11 49.05,44.46 C13.2
  Top 0.3: IC1.29 40.2,67.81 39.1,66.71 C5.2 | C2.1 51.89,85 C1.1 | v31.5,62.21 31.5,64.31 32.45,65.26 | IC1.6 59.8,68.61 v60.1,68.91 60.85,68.16 C3.2
  Top 0.4: 59.4,57.41 59.4,57.11 60.05,56.46 60.7,56.46 | v25.7,80.11 25.66,80.07 R17.2 | JP1.13 80.7,125.25 80.7,123.71 81.06,123.35 R3.2 82.29,122.42 84.7,120.01 85.05,119.66 LED1.C 85.05,117.06 86,116.11 v86,115.31 | v95.9,117.91 96.7,117.11 98,117.11 | R14.2 80.26,83.42 VBAT100.- 80.26,83.85 81.8,82.31 82.79,81.32 U$9.4 | 69.56,59.82 64.88,59.82 64.63,59.82 62.94,59.82 61.86,58.75 61.86,57.43 R21.2 61.6,56.81 61.25,56.46 60.7,56.46 | 69.56,59.82 69.71,59.82 70.02,59.82 71.41,58.44 71.41,57.67 70.81,57.07 IC5.P$1 | IC5.P$5 67.6,51.06 67.6,48.41 65.45,46.26 C10.2 65.45,46.27 65.45,46.53 64.48,47.5 62.01,47.5 60.95,48.57 C19.1 60.95,56.21 60.7,56.46 | 72.7,67.64 72.7,62.97 69.56,59.82
  Top 0.406: JP1.19 82.12,134.6 U$1.3 | v13.6,87.31 13.1,87.81 12.4,87.81 11.84,88.37 T1.E | v68.1,45.41 67.7,45.01 65.45,45.01 | v80.4,40.41 78.06,42.75 2.1 78.06,45.4 C11.2 | C14.1 23.13,45.05 C12.1
  Top 0.8: UEXT.2 12.98,15.43 7.4,21.01 | 7.4,21.01 2,21.01 2,20.81 2.1,20.71 | C14.1 19.49,41.51 16.3,41.51 7.4,32.61 7.4,21.01 | JP2.3 JP3.3 | v81.1,25.51 96.6,25.51 98,26.91 | 98,117.11 98,120.01 | 98,120.01 98,129.11 97.9,129.21 USB1.GND@3 | USB1.GND@1 97.8,120.21 98,120.01
  Top 0.813: C10.2 65.54,45.51 | C11.2 78.06,45.51
  Top 1: 1.1 65.45,42.76 65.45,45.01 C10.2 | 2.5,129.31 arc-84 98,129.11 | 2.5,129.11 2,128.61 2,123.31 2,21.01 2,20.61 arc85 98,20.11 98,26.91 98,117.11 | VBAT100.- 83.3,91.41 97.9,91.41 | 78.06,45.51 79.71,47.16 C18.2
  Bottom 0.2: v50.9,80.01 52,81.11 v52,87.31 | v34,47.71 25.4,47.71 24.2,46.51 v24.2,46.21 | v58,57.01 57.5,57.01 56.5,57.01 54.85,55.36 v54.85,55.21 | v47.6,66.11 47.6,67.21 49.8,69.41 v49.8,71.51 | v66.1,70.81 67.1,69.81 v71.1,69.81 75,73.71 v75,80.71
  Bottom 0.3: v60.1,68.91 60.1,72.31 59.8,72.61 v59.1,73.31
  Bottom 0.4: v89.3,125.81 90.7,124.41 95.8,124.41 96.6,123.61 96.6,120.21 95.9,119.51 v95.9,117.91 96.7,117.11 96.7,113.61 96.05,112.96 BAT_CH.2 88.9,110.81 85.2,110.81 84,112.01 84,113.31 v86,115.31 | v25.7,80.11 29.7,76.11 29.7,65.91 29.7,64.01 v31.5,62.21
  Bottom 0.406: JP2.3 21.7,100.26 21.7,88.31 20.7,87.31 18.1,87.31 | 18.1,87.31 v13.6,87.31 | v25.7,80.11 20.3,85.51 20.3,85.91 18.9,87.31 18.1,87.31 | v80.4,40.41 73.1,40.41 v68.1,45.41
  Bottom 0.8: JP5.10 44.92,36.59 46.6,34.91 52.44,34.91 JP8.2 71.92,19.83 77.6,25.51 v81.1,25.51
  Bottom 1: JP1.19 78.97,131.94 79,131.91
  Bottom 1.27: JP8.1 JP8.2 | JP1.20 JP1.19 JP1.17 JP1.18 JP1.16 JP1.15 JP1.13 | JP1.13 JP1.14 | JP1.13 76.4,126.98 76.4,129.41 79,129.41 79,131.91 79,132.01 76.5,132.01 76.5,134.71
  pour Top (isolate 1.27): 94,56.01 94,65.51 51.8,65.51 51.8,20.01 100.1,20.01 100.1,58.91 103.2,58.91 103.2,-1.39 0,-1.39 0,149.11 100.7,149.11 100.7,60.41 98.6,60.41 98.6,56.01
  pour Bottom (isolate 1.27): 0,144.61 0,-0.39 105,-0.39 105,149.61 0,149.61
INT0-BUTTON1  (via drill 0.35, 0.4)
  Top 0.2: 12.3,117.61 12.27,117.64 A.3 12.2,118.51 12.7,119.01 13.5,119.81 v14.6,119.81 | v29.8,87.71 29.8,87.61 35,82.41 39.6,82.41 43,79.01 43,74.51 44,73.51 45,73.51 45.3,73.51 46.3,72.51 48,70.81 48,69.51 51.6,65.91 51.9,65.91 53.2,64.61 IC1.43 53.3,62.41 v53.3,60.71 | v53.1,55.11 53.8,54.41 54.9,54.41 56,53.31 56,51.41 55.7,51.11 v55.7,50.81 | IC3.8 52.31,45.59 53.14,44.76 v54.15,44.76
  Top 0.406: A.3 A.4
  Bottom 0.2: v29.8,87.71 29.3,88.21 29.3,103.61 27.5,105.41 27.5,115.21 23.6,119.11 22.9,119.81 v14.6,119.81 | v53.3,60.71 53.1,60.51 v53.1,55.11 | v55.7,50.81 55.1,50.21 55.1,46.64 55.1,45.72 v54.15,44.76
INT2
  Top 0.2: IC1.2 62.7,65.41 65.01,67.72 IC2.6
INT3-BUTTON2  (via drill 0.35, 0.4)
  Top 0.2: v25.9,115.41 24,117.31 B.3 | IC1.32 42.2,65.41 39.2,62.41 v39.2,62.11
  Top 0.4: B.4 B.3 | v41.7,53.71 45.36,53.71 IC3.1 IC3.2
  Bottom 0.2: v25.9,115.41 25.9,105.61 28.5,103.01 28.5,87.71 28.6,87.61 30.7,85.51 30.7,75.41 30.7,75.4 30.7,74.61 38.45,66.86 38.45,64.73 39.2,63.98 39.2,62.6 v39.2,62.11 40,62.91 40.4,62.91 41.2,62.91 41.5,62.61 43,61.11 43,59.91 43,55.01 v41.7,53.71
INT4
  Top 0.2: IC1.3 62.7,66.21 66.1,69.61 IC2.4
MCLR  (via drill 0.35)  (2 unrouted)
  Top 0.2: 49.3,74.61 IC1.18 49.2,81.01 47.1,83.11 46.5,83.11 | C2.2 R12.2 44.2,83.11 43,83.11 36,83.11 31.2,87.91 29.4,89.71 v18.1,89.71 | ICSP.6 12.9,127.91 12.1,127.11
  Top 0.406: RESET.3 RESET.4
  Bottom 0.2: v18.1,89.71 12.9,94.91 ICSP.6
N$1
  Top 0.2: IC1.11 57.5,72.61 58.2,73.31 58.2,76.71 58.7,77.21 R18.1 | R18.1 | R18.1 59.81,77.22 R13.2
  Top 0.4: R18.1
N$3
  Top 0.3: IC1.7 58.4,69.41 59.1,70.11 62.44,70.11 C3.1
N$5
  Top 0.2: 69.25,54.59 69.51,54.85 IC5.P$3
  Top 0.4: C17.2 66.27,54.59 69.25,54.59 72.67,54.59 R19.2
N$6
  Top 0.4: LED1.A 82.95,115.16 R7.2
N$7  (1 unrouted)
  Top 0.2: 17.2,108.81 14.2,105.81 14.2,99.41 16.2,97.21 16.2,51.81 18.1,50.11 29.5,50.11 33.7,45.91 39.8,45.91 40.9,45.91 41.6,46.61 41.6,48.11 44.3,50.81 45.65,50.81 IC3.3
N$8
  Top 0.2: LED2.A 13,104.07 13,98.51 15.1,96.41 15.1,51.01 17,49.11 28.7,49.11 32.9,44.91 40.6,44.91 41.2,44.91 42.2,45.91 42.2,47.81 44,49.61 45.65,49.61 IC3.4
N$14
  Top 0.2: R10.2 13.4,81.2 13.4,51.21 16.5,48.11 28.4,48.11 32.2,44.31 41,44.31 41.7,44.31 42.8,45.41 42.8,47.41 43.7,48.31 IC3.5
N$15
  Top 0.2: LED3.C 17.72,110.83 R9.2
N$16
  Top 0.2: LED2.C 8.68,110.93 10.8,108.81 11.22,108.81 R8.2
N$17
  Top 0.2: R10.1 T1.B
N$18
  Top 0.2: ICSP.3 R1.2
N$19
  Top 0.2: ICSP.2 23.11,134.24 R2.2
N$20
  Top 1: VBAT101.- VBAT100.+
N$22
  Top 0.2: A.2 3.5,115.54 3.5,119.01 5.11,120.62 R6.2
  Top 0.406: A.1 A.2
N$23
  Top 0.2: B.2 14.9,115.94 14.9,117.91 17.99,121 R5.2
  Top 0.406: B.1 B.2
N$24
  Top 0.4: U$1.4 87.4,126.51 R4.1
N$25
  Top 0.4: U$1.6 82.29,128.71 R3.1
N$26  (1 unrouted)
  Top 0.2: T1.C 10.21,92.6 10.2,92.6 SG1.+ | 7,95.81 7.2,95.81
N$27  (via drill 0.6)
  Top 0.4: IC5.P$8 70.85,52.28 73.1,52.28 77.93,52.28 L1.1 83.52,52.64 v83.57,52.59 | C17.1 66.17,52.73 66.17,51.51 66.17,50.15 v66.07,50.04
  Top 1: U$12.A 78.29,51.05 L1.1
  Bottom 0.4: v83.57,52.59 83.57,47.81 83.57,46.73 80.49,43.65 72.18,43.65 68.94,46.89 66.07,49.76 v66.07,50.04
N$28  (via drill 0.6)  (1 unrouted)
  Top 0.4: U$1.2 84.9,135.81 84.1,136.61 83.5,137.21 79.1,137.21 77.3,139.01 v71.9,139.01 | v71.7,59.81 78.9,67.01 82.2,67.01 83.2,68.01 v83.2,69.41 | IC5.P$2 70.17,56.43 70.17,57.67 69.25,58.59 v67.71,58.59
  Bottom 0.4: v71.9,139.01 70.6,137.71 70.6,93.61 67.3,90.31 67.3,87.01 71.6,82.71 78.3,82.71 84.2,76.81 84.2,70.01 83.6,69.41 v83.2,69.41 | 75.8,64.01 77.1,65.31 | v71.7,59.81 70.48,58.59 v67.71,58.59
N$29
  Top 0.4: R20.2 63.86,54.7 63.94,54.78 R21.1 64.52,57.25 64.78,57.51 68.17,57.51 68.86,56.83 IC5.P$4
N$30  (via drill 0.6, 1)
  Top 0.4: IC5.P$6 IC5.P$7 70.16,50.2 U$12.C 68.69,48.91 v68.66,48.88 | R20.1 63.86,52.72 63.87,52.7 v63.87,51.07
  Top 0.8: v68.63,42.73 71.45,45.55 U$12.C | v68.17,34.41 68.67,33.92 F1.P$1
  Bottom 0.4: v63.87,51.07 63.91,51.11 66.9,51.11 68.66,49.34 v68.66,48.88
  Bottom 0.8: v68.17,34.41 71.41,37.65 71.41,39.34 71.41,39.96 v68.63,42.73
N$36
  Top 0.2: R16.2 81.8,76.79 81.8,74.21 82.13,73.88 U$9.1
N$37
  Top 0.2: R15.2 17.2,75.81 17.2,75.51 17.25,75.51 U$8.1
N$38
  Top 0.2: U$9.3 77.11,75.86 R14.1
N$39
  Top 0.152: IC1.30 43.65,66.99 43.65,67.01
  Top 0.3: 31.3,58.71 32.8,58.71 41.1,67.01 43.65,67.01 IC1.30 44.1,67.01 | 31.3,58.71 30.8,58.71 30.7,58.71 | C8.2 31.3,55.44 31.3,58.71
  Top 0.4: CRYSTAL.2 30.79,58.72 30.8,58.71
N$40
  Top 0.2: R17.1 21.6,76.36 21.6,74.21 21.92,73.89 U$8.3
N$41
  Top 0.2: CRYSTAL.1 40.41,57.78 40.41,56.96 C9.2
  Top 0.3: IC1.31 41.8,66.21 37.9,62.31 37.9,58.71 | CRYSTAL.1 39.4,58.72
  Top 0.4: 37.9,58.71 39.39,58.71 39.4,58.72
N$42  (via drill 0.35)
  Top 0.2: POT1.1 70.44,76.65 71.1,77.31 73,77.31 73.7,76.61 POT1.2 74.6,73.88 U$9.2 | POT1.1 70.4,75.75 70.4,75.71 | v69.3,74.91 70.18,75.79 POT1.1 | v69.3,71.11 69.3,69.7 IC2.3
  Bottom 0.2: v69.3,71.11 v69.3,74.91
N$44
  Top 0.152: R11.1 55.08,83.5 52.54,83.5 C1.2
  Top 0.2: IC1.17 50,80.81 51.94,82.75 C1.2 51.98,83.11 55.3,83.11
N$45  (via drill 0.4)
  Top 0.2: U$8.2 23.42,74.64 POT.2 | IC2.1 70.3,66.8 70.3,66.31 70.3,65.11 67,61.81 63.7,61.81 62.1,63.41 55,63.41 54.7,63.71 53.8,64.61 53.8,65.81 53.1,66.51 51.8,66.51 48.9,69.41 v48.9,70.21 | v26.5,69.71 26.31,69.9 26.31,73.91 | v44.5,62.71 43.7,61.91 v40.9,61.91
  Top 0.4: POT.1 28.73,72.81 26.9,72.81 26.31,73.4 26.31,73.91 POT.2
  Bottom 0.2: v48.9,70.21 44.5,65.81 v44.5,62.71 | v26.5,69.71 26.5,57.51 28.7,55.31 33.4,55.31 33.6,55.31 34.3,55.31 v40.9,61.91
PMA3  (via drill 0.35)
  Top 0.2: v49.2,59.51 IC1.38 | v22.8,43.11 22.7,43.01 22.7,42.01 23.04,41.67 IC4.P$2
  Bottom 0.2: v49.2,59.51 49.2,54.81 43.3,48.91 24.9,48.91 23.1,47.11 22.8,46.81 v22.8,43.11
PMA4  (via drill 0.35)
  Top 0.2: IC4.P$3 22.4,41.01 v22.2,40.81 | v48.4,60.21 IC1.37
  Bottom 0.2: v48.4,60.21 48.4,55.31 42.8,49.71 24.6,49.71 22.3,47.41 22,47.11 22,41.61 22,40.81 v22.2,40.81
PMA7  (via drill 0.35, 0.4)
  Top 0.2: 29.44,41.67 IC4.P$15 31.26,41.67 31.6,42.01 31.6,43.11 v30.2,44.51 | IC1.13 v53.2,76.41 53.2,77.61 52.1,78.71 v52.1,79.61 | v51.5,93.61 50.9,94.21 50.9,100.01 49.8,101.11 45.8,105.11 40.1,105.11 24.8,120.41 v24.8,124.11 | v26,127.91 25.2,128.71 R2.1
  Bottom 0.2: v53.2,76.41 53.2,71.81 50.6,69.21 50.6,55.21 44,48.61 43.8,48.41 38.8,48.41 34.9,44.51 v30.2,44.51 | v52.1,79.61 52.7,80.21 52.7,88.71 52.7,92.41 v51.5,93.61 | v24.8,124.11 26,125.31 v26,127.91
PMA10  (via drill 0.35)
  Top 0.2: IC4.P$14 | IC1.12 v54,77.51 53.4,78.11 v53.4,81.31 | v53.4,94.71 53.4,101.01 52.5,101.91 48,106.41 40.8,106.41 26.2,121.01 26.2,125.01 25.4,125.81 23,125.81 22.8,125.81 20.51,128.1 R1.1 | IC4.P$14 31.4,41.01 31.8,41.41 v32.8,41.41
  Bottom 0.2: v54,77.51 54,71.51 51.4,68.91 51.4,68.61 51.4,55.31 50.7,54.61 44,47.91 42.5,47.91 42.45,47.86 35.9,41.31 35.9,39.71 35.3,39.11 32.7,39.11 32.4,39.41 32.4,41.01 v32.8,41.41 | v53.4,94.71 v53.4,81.31
QD  (via drill 0.35)
  Top 0.2: 49.4,45.41 49.6,45.21 v49.6,44.91
  Top 0.254: 48.95,45.86 47.77,47.03 IC3.6
  Top 0.3: 48.95,45.86 49.4,45.41
  Bottom 0.2: v49.6,44.91 50.75,44.91 JP5.1
QE
  Top 0.152: JP5.2 55.08,37.78 55.1,37.91
  Top 0.3: 57.3,42.91 57.3,45.21 54.3,48.21 52.41,48.21 IC3.10
  Top 0.305: 57.3,42.91 57.3,40.11 55.1,37.91
QF
  Top 0.3: 58.1,43.51 58.1,45.61 54.6,49.11 54.13,49.57 IC3.11
  Top 0.305: 58.1,43.51 58.1,39.11 55.4,36.41 54.8,36.41 53.8,37.41 53.8,39.32 JP5.3
QG
  Top 0.152: JP5.4 52.54,37.78 52.57,37.64
  Top 0.3: 58.9,43.71 58.9,45.91 55.3,49.51 54.7,50.11 54.7,50.71 54.56,50.84 IC3.12
  Top 0.305: 52.57,38.04 52.57,37.64 54.8,35.41 55.5,35.41 58.9,38.81 58.9,43.71
QH
  Top 0.254: 50.4,47.01 50.4,51.41 51.1,52.11 IC3.13
  Top 0.3: JP5.5 50.4,40.98 50.4,47.01
RPB9  (via drill 0.35, 0.6)
  Top 0.2: v58.4,64.71 58.3,64.61 IC1.1
  Top 0.4: v94.7,114.81 95.6,113.91 95.6,107.91 95.6,105.71 v88.2,98.31 | v80.5,29.61 83.5,29.61 88.2,34.31 88.2,78.21 88.2,87.21 v87.3,88.11 | v89.9,132.11 87.69,134.32 U$1.1
  Top 0.406: U$1.1 87.4,134.11 87.3,134.01
  Bottom 0.2: JP5.6 50,38.01 51.6,36.41 53.8,36.41 55,36.41 66.7,36.41 66.9,36.61 69.1,38.81 69.1,40.21 67.9,41.41 64.2,45.11 60.3,49.01 60.3,59.51 58.4,61.41 v58.4,64.71
  Bottom 0.4: v89.9,132.11 87.9,130.11 87.9,124.51 94.1,118.31 94.7,117.71 v94.7,114.81 | v87.3,88.11 87.3,97.41 v88.2,98.31
  Bottom 0.406: v80.5,29.61 79.48,29.61 72.5,22.62 67.58,22.62 53.8,36.41
SCK1  (via drill 0.35)
  Top 0.2: v52.4,77.11 IC1.14 52.4,69.21 v53.2,68.41
  Bottom 0.2: v52.4,77.11 60.45,85.16 60.45,94.81 JP4.25 | UEXT.9 29.5,14.31 29.5,16.71 28.5,17.71 28.5,24.91 28.5,26.11 32.9,30.51 32.9,35.21 33.7,36.01 33.8,36.11 36,36.11 52,52.11 54.26,52.11 | v53.2,68.41 54,68.41 57.6,64.81 57.6,61.21 59.5,59.31 59.5,58.61 59.5,55.91 58.2,54.61 57.68,54.09 56.54,54.09 54.56,52.11 54.26,52.11 | 54.26,52.11 54.7,52.11
  Bottom 1.27: JP4.26 JP4.25
SCL2  (via drill 0.3, 0.35)
  Top 0.152: v16.98,77.15 16.98,93.66 37.3,93.66 39.84,96.2 JP4.7
  Top 0.2: IC1.24 41.8,71.81 v40.75,72.86
  Top 0.3: 40.7,72.91 40.6,73.01 38.7,73.01 37.8,73.01 21.6,56.81 21.4,56.61 21.4,52.71 v21.3,52.61
  Bottom 0.152: v16.98,77.15 16.98,55.56 15.71,55.56 10.63,50.48 10.63,12.38 15.71,12.38 16.98,11.11 22.06,11.11 23.33,12.38 UEXT.5
  Bottom 0.2: v40.75,72.86 34.25,79.36 34.25,87.11 35,87.86 36,87.86 39.42,91.28 JP4.7 | 14.5,22.11 15.3,21.31 16.9,21.31 21.7,16.41 21.7,14.09 UEXT.5
  Bottom 0.3: 14.5,22.11 14.5,48.81 18.3,52.61 v21.3,52.61
  Bottom 1.27: JP4.8 JP4.7
SDA2  (via drill 0.35)
  Top 0.2: IC1.23 42.75,72.61 v41.5,73.86
  Top 0.3: v41.5,73.86 37.55,73.86 20.5,56.81 20.3,56.61 v20.3,51.01
  Bottom 0.2: v41.5,73.86 35,80.36 35,86.61 35.5,87.11 37,87.11 41.96,92.07 JP4.9 | 15.7,22.61 17.1,22.61 23,16.71 UEXT.6
  Bottom 0.3: 15.7,22.61 15.7,48.21 18.5,51.01 v20.3,51.01
  Bottom 1.27: JP4.10 JP4.9
SDI1  (via drill 0.35, 0.4)
  Top 0.2: v52.2,59.41 51.6,60.01 IC1.41 51.6,64.81 v46.1,70.31 | v49.4,92.91 49.6,92.71 61.7,92.71 62.4,93.41 66.7,93.41 67.36,94.07 JP4.29
  Bottom 0.2: UEXT.8 24.54,16.43 24.54,26.55 22.2,28.89 22.2,32.21 24.1,34.11 28.3,38.31 35.4,38.31 52.2,55.11 52.2,56.21 v52.2,59.41 | v46.1,70.31 49.4,73.61 v49.4,92.91
  Bottom 1.27: JP4.30 JP4.29
SDO1  (via drill 0.35, 0.4)
  Top 0.2: IC1.44 54.4,62.11 v54.4,60.71 55.4,60.71 55.8,61.11 62.2,61.11 67.8,61.11 v69.6,62.91 | v78.7,70.61 78.7,69.41 v74.8,65.51
  Bottom 0.2: UEXT.7 26.8,14.15 26.8,16.21 25.8,17.21 25.8,25.91 30,30.11 30,35.71 32,37.71 35.7,37.71 52,54.01 53.2,54.01 54,54.81 54,55.11 54,60.31 v54.4,60.71 | JP4.27 64.82,95.83 62.1,93.11 61.5,92.51 61.5,86.01 62.7,84.81 62.8,84.71 63.8,84.71 65.1,83.41 65.1,76.81 65.8,76.11 70.1,76.11 73.3,79.31 73.3,80.51 74.6,81.81 75.3,81.81 | v74.8,65.51 72.2,62.91 v69.6,62.91 | 75.3,81.81 75.6,81.81 | v78.7,70.61 77.5,71.81 77.5,79.91 75.6,81.81 | 75.6,81.81 75.3,81.81
  Bottom 1.27: JP4.28 JP4.27
U1RX  (via drill 0.35)
  Top 0.3: v45.4,59.61 46,60.21 IC1.34
  Bottom 0.2: UEXT.4 20.46,16.15 16.5,20.11 14.9,20.11 13.2,21.81
  Bottom 0.3: 13.2,21.81 13.2,49.51 17.4,53.71 24.8,53.71 27.3,51.21 41.9,51.21 43.4,52.71 44.5,53.81 44.5,54.41 44.5,58.71 v45.4,59.61
U1TX  (via drill 0.35)
  Top 0.3: v41.7,63.51 42.8,64.61 IC1.33
  Bottom 0.2: 11.8,21.51 14.3,19.01 16.4,19.01 19.2,16.21 19.2,14.15 UEXT.3
  Bottom 0.3: 11.8,21.51 11.8,50.41 16.15,54.76 25.45,54.76 27.9,52.31 41.7,52.31 43.15,53.76 43.7,54.31 43.7,55.11 43.7,61.51 v41.7,63.51
U2RX_D  (via drill 0.35)
  Top 0.2: v57.7,85.81 57.7,79.41 v56.4,78.11 | v58.2,67.01 IC1.4 56.7,67.01 56.8,67.11
  Bottom 0.2: JP4.21 57.2,86.31 v57.7,85.81 | v56.4,78.11 56.4,70.81 56.4,68.81 v58.2,67.01 58.5,66.71 60.5,66.71 61.1,66.71 62.6,68.21 80.1,68.21 81.6,66.71 85,63.31 85,18.35 JP8.10
  Bottom 1.27: JP4.22 JP4.21
U2TX_D  (via drill 0.35)
  Top 0.2: v56.7,85.11 56.7,79.81 56.5,79.81 55.2,78.51 55.2,77.61 55.5,77.31 55.7,77.11 v57.1,77.11 | v59.4,67.71 56.1,67.71 | 56.1,67.71 56,67.81 | 56.1,67.71 IC1.5
  Bottom 0.2: JP4.19 54.66,87.15 v56.7,85.11 | JP8.9 86.2,17.01 86.2,63.41 81.9,67.71 80.7,68.91 61.8,68.91 60.6,67.71 v59.4,67.71 58.9,67.71 58.6,67.71 57.3,69.01 57.3,76.91 v57.1,77.11
  Bottom 1.27: JP4.20 JP4.19
USB_D+
  Top 0.2: IC1.8 58.2,70.21 62.9,74.91 62.9,78.91 88.7,104.71 88.7,124.11 89.1,124.51 89.3,124.71 USB1.D+
USB_D-
  Top 0.2: IC1.9 58.1,71.01 61.5,74.41 61.5,78.61 88.1,105.21 88.1,126.21 89.1,127.21 92.6,127.21 93.3,127.91 93.6,128.21 94.7,128.21 95.3,127.61 95.3,125.81 93.4,123.91 USB1.D-
VBAT  (via drill 0.6, 1, 1.2)
  Top 0.4: U$1.5 84.1,128.02 84.1,122.11 86.7,119.51 v86.7,119.21 | R13.1 63.14,81.45 64.6,82.91 69.8,88.11 v69.8,89.71
  Top 0.8: v86.3,112.61 79.3,105.61 v79.2,105.61
  Top 1: VBAT101.+ 29.4,91.41 29.5,91.31 30.5,91.31 32.2,89.61 63.4,89.61 69.7,89.61 v69.8,89.71 | v86.3,66.41 86.3,62.71 | 86.3,62.71 81.23,57.64 78.95,57.64 | 78.95,57.64 L1.2 | C18.1 80.21,49.04 84.19,49.04 86.3,51.16 86.3,62.71 | R19.1 73.88,57.64 78.95,57.64
  Bottom 0.4: v86.7,119.21 90.95,114.96 BAT_CH.1 88.65,114.96 v86.3,112.61
  Bottom 0.8: JP8.3 77.74,9.61 82.6,9.61 88.4,15.41 88.4,71.61 86.2,73.81 | 77.3,89.71 77.3,97.81 77.3,103.71 v79.2,105.61
  Bottom 1: v69.8,89.71 77.3,89.71 86.2,80.81 86.2,73.81 86.2,66.51 v86.3,66.41

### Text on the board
tNames: MINI BREADBOARD | BASEBOT
_tplace: + | + | +
_bplace: + | - | + | - | - | + | - | +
